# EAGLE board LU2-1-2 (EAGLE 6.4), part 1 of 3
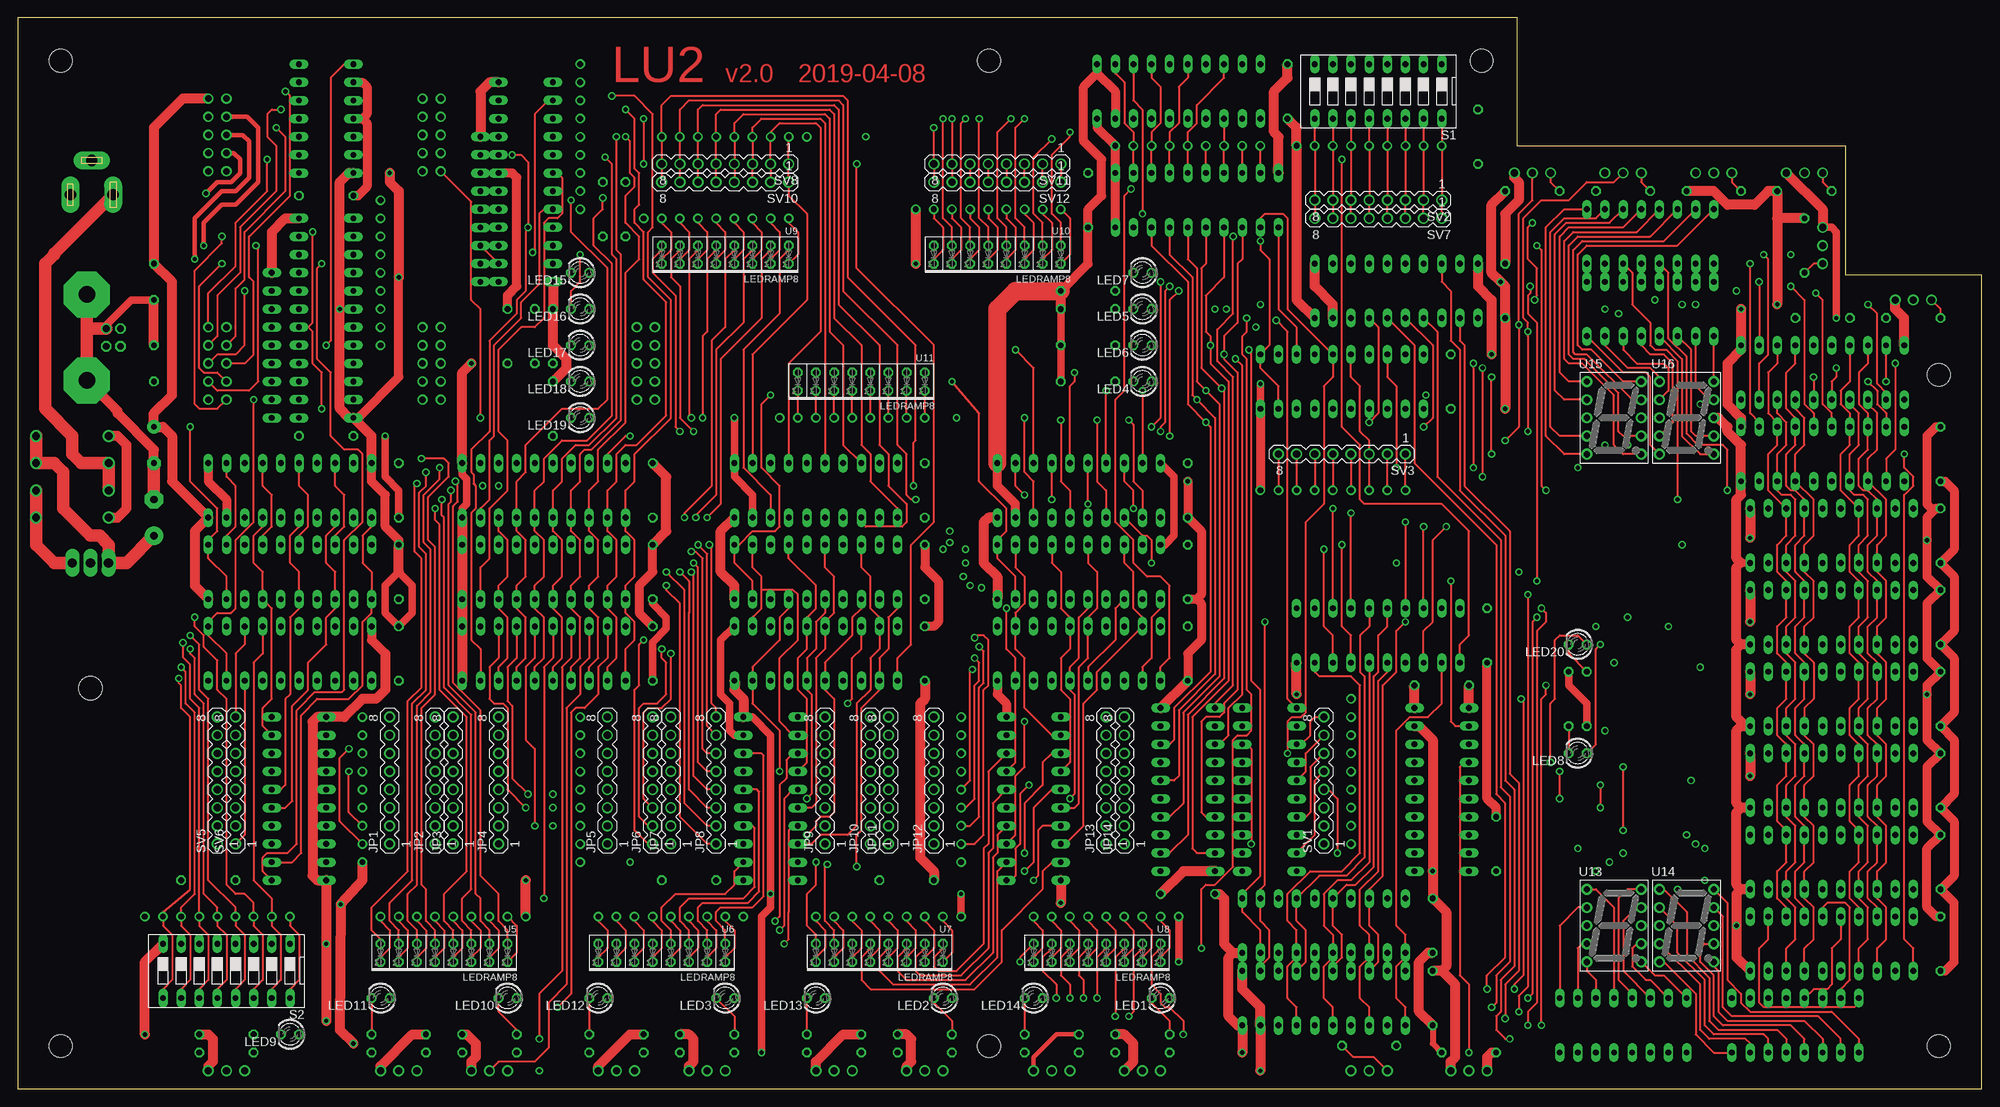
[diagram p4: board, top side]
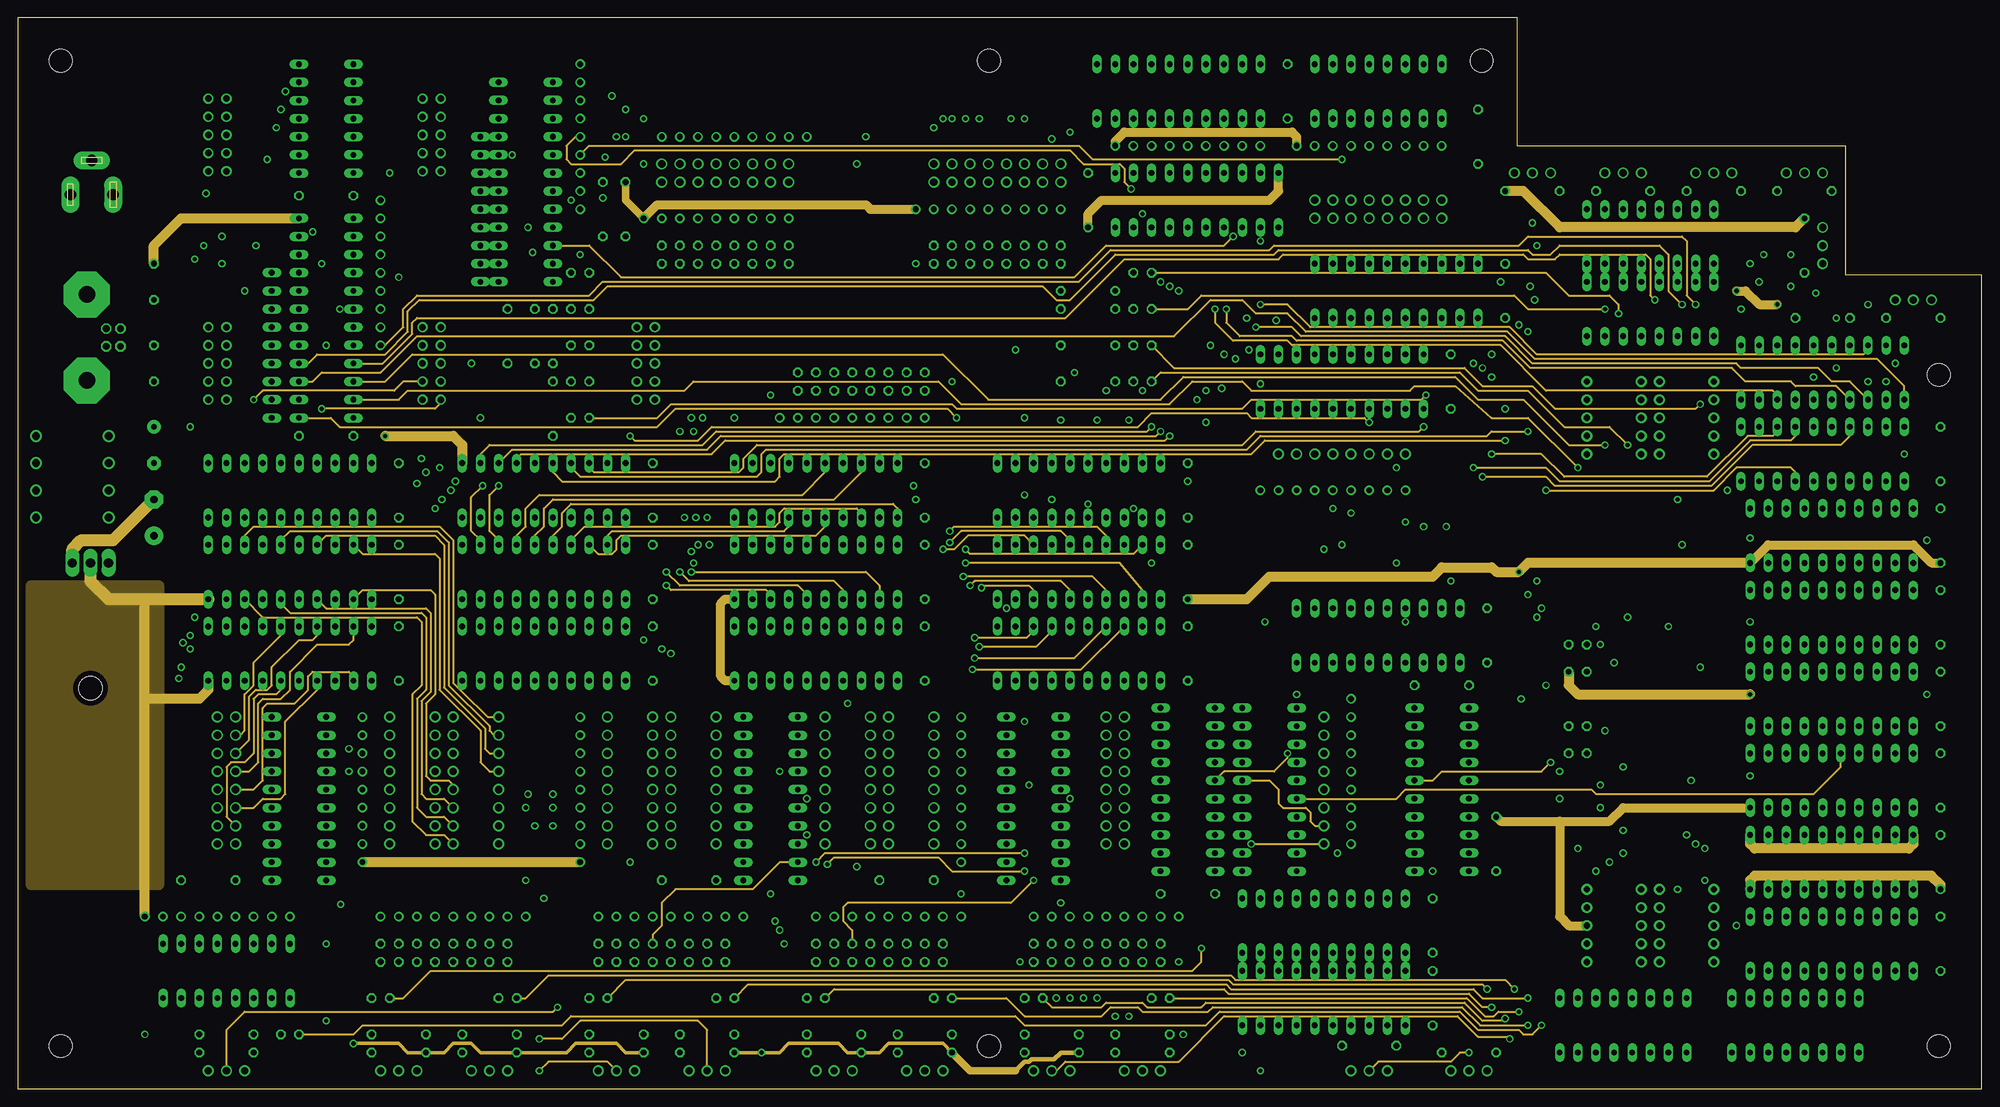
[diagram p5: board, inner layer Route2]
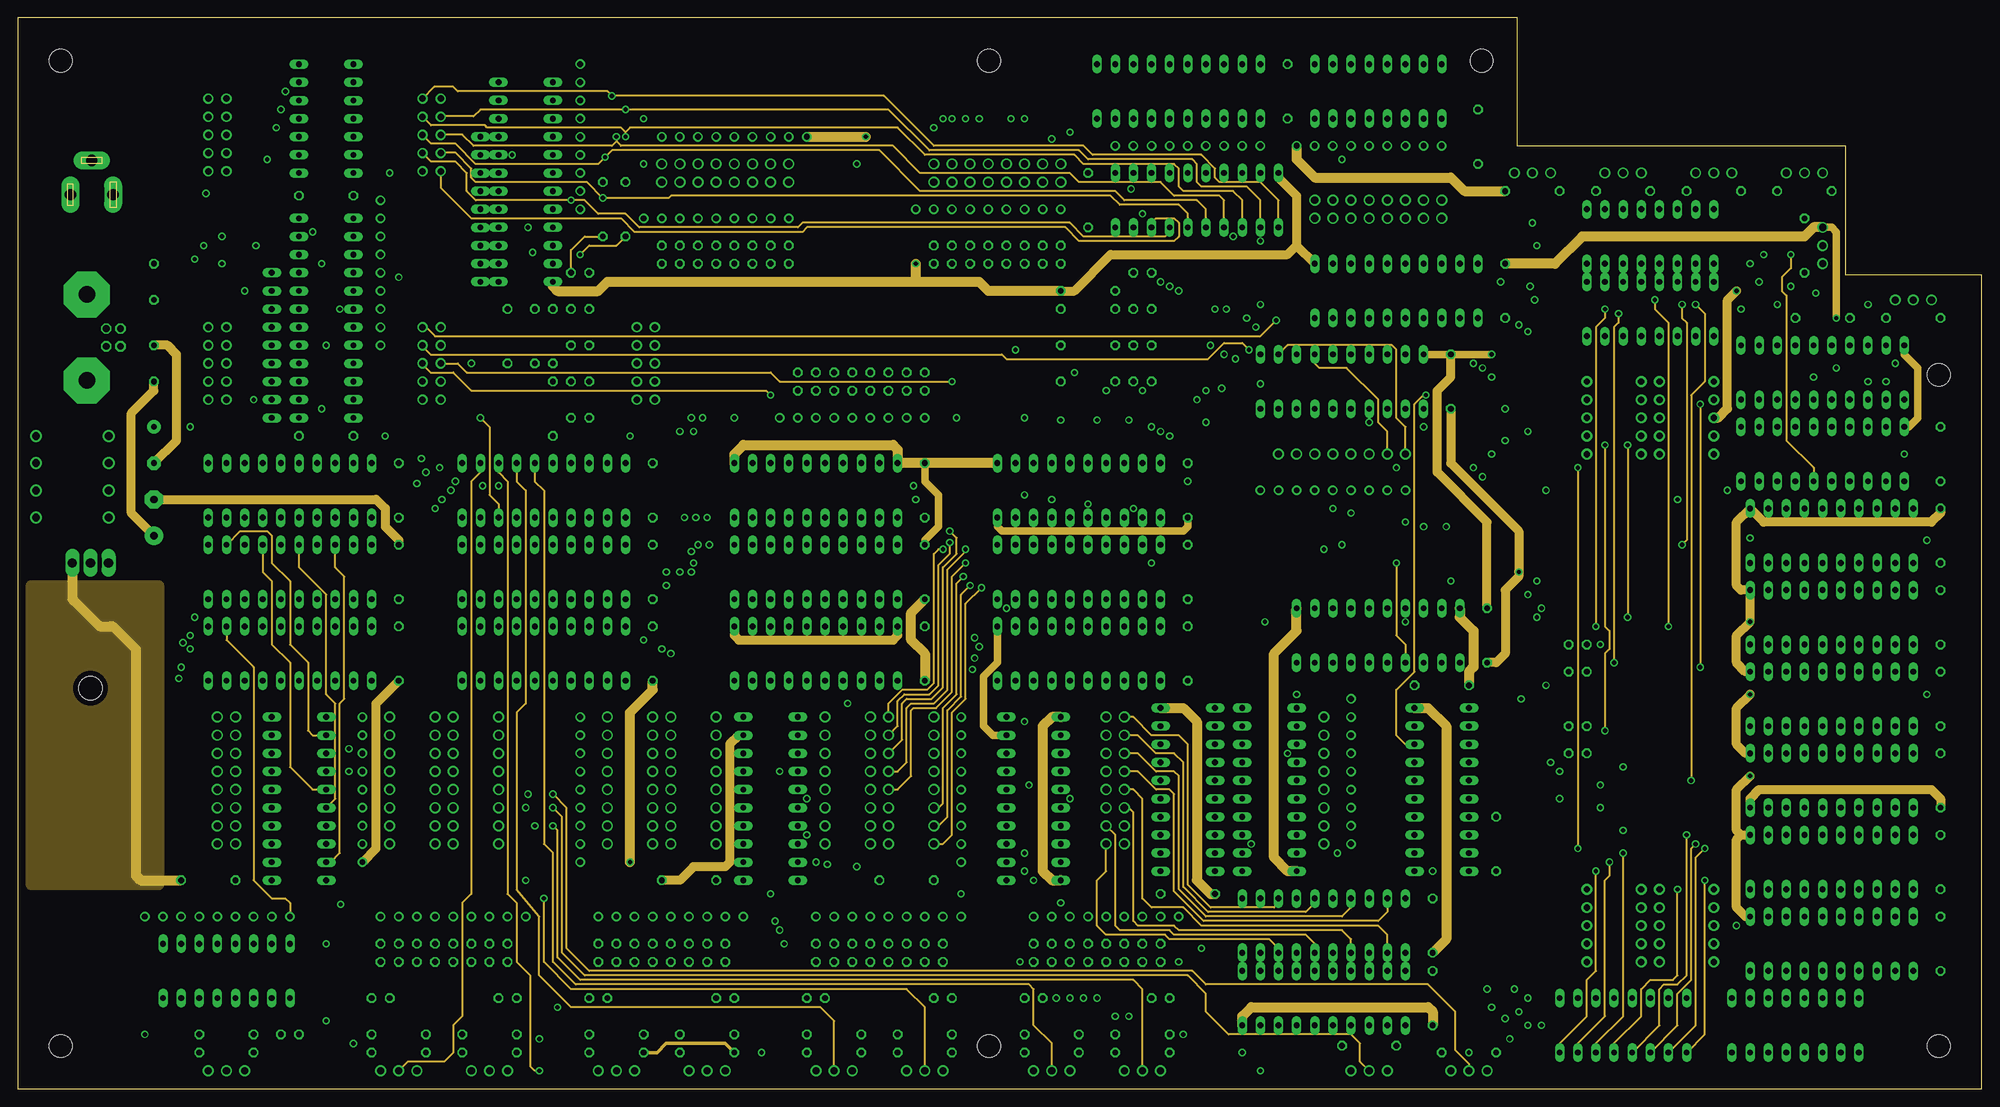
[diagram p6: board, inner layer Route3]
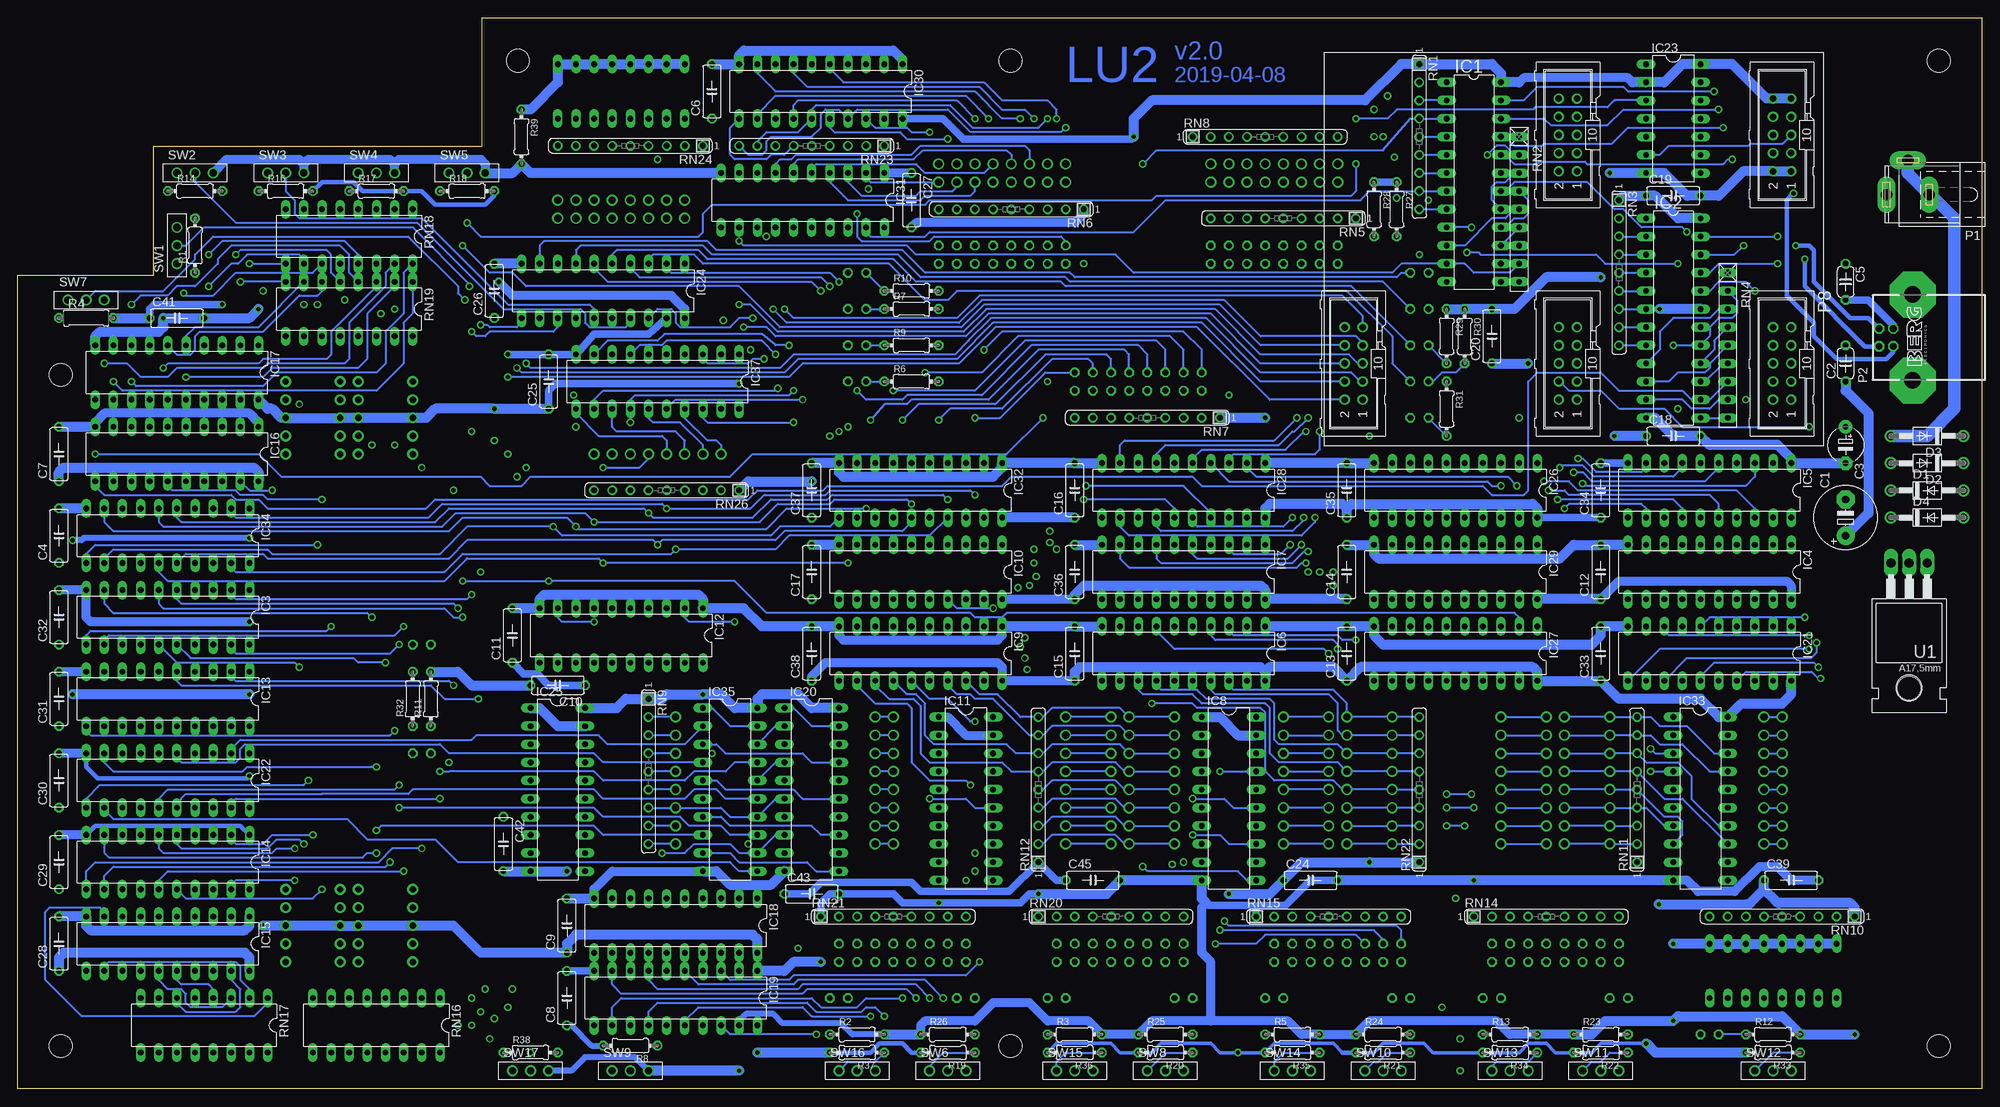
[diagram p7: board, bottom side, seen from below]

Size 275 x 150 mm. Coordinates in mm from the lower left corner, seen from the top.
Outline: 0,0 275,0 275,114 256,114 256,132 210,132 210,150 0,150 0,0
Copper layers (1+2*3+16): Top 0.035mm / dielectric 0.3mm / Route2 0.035mm / dielectric 0.9mm / Route3 0.035mm / dielectric 0.3mm / Bottom 0.035mm
Design rules "default *": minimum track width 10mil, minimum drill 22mil, track to track 10mil, track to pad 10mil, pad to pad 10mil, via to via 10mil, smd to smd 8mil, copper to edge 30mil, drill to drill 8mil, minimum pad ring 10mil, minimum via ring 8mil, stop-mask expansion 4mil, vias tented up to drill 0mil, thermal gap 10mil
Holes 3.2 mm at 6,6 6,144 205,144 269,6 136,6 136,144 269,100
tKeepout: area 0,27.9 to 20.3,71.1

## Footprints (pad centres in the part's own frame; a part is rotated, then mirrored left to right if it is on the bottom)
E5-8,5 = drill 1.016 pad 2.54: + -2.54,0 | drill 1.016 pad 2.54 octagon: - 2.54,0
C050-024X044 = drill 0.813 octagon: 1 -2.54,0; 2 2.54,0
E5-5 = drill 0.813 pad 1.905: + -2.54,0 | drill 0.813 pad 1.905 octagon: - 2.54,0
C313 = drill 0.813 octagon: 1 -3.81,0; 2 3.81,0
DO41-10 = drill 1.118: A 5.08,0; C -5.08,0
DIL24-3 = drill 0.813 long: 1 -13.97,-3.81; 2 -11.43,-3.81; 3 -8.89,-3.81; 4 -6.35,-3.81; 5 -3.81,-3.81; 6 -1.27,-3.81; 7 1.27,-3.81; 8 3.81,-3.81; 9 6.35,-3.81; 10 8.89,-3.81; 11 11.43,-3.81; 12 13.97,-3.81; 13 13.97,3.81; 14 11.43,3.81; 15 8.89,3.81; 16 6.35,3.81; 17 3.81,3.81; 18 1.27,3.81; 19 -1.27,3.81; 20 -3.81,3.81; 21 -6.35,3.81; 22 -8.89,3.81; 23 -11.43,3.81; 24 -13.97,3.81
DIL20 = drill 0.813 long: 1 -11.43,-3.81; 2 -8.89,-3.81; 3 -6.35,-3.81; 4 -3.81,-3.81; 5 -1.27,-3.81; 6 1.27,-3.81; 7 3.81,-3.81; 8 6.35,-3.81; 9 8.89,-3.81; 10 11.43,-3.81; 11 11.43,3.81; 12 8.89,3.81; 13 6.35,3.81; 14 3.81,3.81; 15 1.27,3.81; 16 -1.27,3.81; 17 -3.81,3.81; 18 -6.35,3.81; 19 -8.89,3.81; 20 -11.43,3.81
DIL14 = drill 0.813 long: 1 -7.62,-3.81; 2 -5.08,-3.81; 3 -2.54,-3.81; 4 0,-3.81; 5 2.54,-3.81; 6 5.08,-3.81; 7 7.62,-3.81; 8 7.62,3.81; 9 5.08,3.81; 10 2.54,3.81; 11 0,3.81; 12 -2.54,3.81; 13 -5.08,3.81; 14 -7.62,3.81
MA08R-1 = drill 1.016: 1 -8.89,0; 2 -6.35,0; 3 -3.81,0; 4 -1.27,0; 5 1.27,0; 6 3.81,0; 7 6.35,0; 8 8.89,0
LED3MM = drill 0.813 octagon: A -1.27,0; K 1.27,0
DC21CLIFF = drill 1.6 pad 2.54 long: 1 0.81,0; 2 3.81,-4.8; 3 6.81,0
1729-S = drill 0.95 octagon: 1 1.25,5.98; 2 -1.25,5.98; 3 -1.25,3.98; 4 1.25,3.98 | drill 2.3 pad 6.452 octagon: S1 -6.02,1.27; S2 6.02,1.27
ARM_CTRL = drill 0.914: 1 5.08,1.27; 2 5.08,-1.27; 3 2.54,1.27; 4 2.54,-1.27; 5 0,1.27; 6 0,-1.27; 7 -2.54,1.27; 8 -2.54,-1.27; 9 -5.08,1.27; 10 -5.08,-1.27; 11 -26.92,1.27; 12 -26.92,-1.27; 13 -29.46,1.27; 14 -29.46,-1.27; 15 -32,1.27; 16 -32,-1.27; 17 -34.54,1.27; 18 -34.54,-1.27; 19 -37.08,1.27; 20 -37.08,-1.27; 21 -26.92,-28.73; 22 -26.92,-31.27; 23 -29.46,-28.73; 24 -29.46,-31.27; 25 -32,-28.73; 26 -32,-31.27; 27 -34.54,-28.73; 28 -34.54,-31.27; 29 -37.08,-28.73; 30 -37.08,-31.27; 31 5.08,-28.73; 32 5.08,-31.27; 33 2.54,-28.73; 34 2.54,-31.27; 35 0,-28.73; 36 0,-31.27; 37 -2.54,-28.73; 38 -2.54,-31.27; 39 -5.08,-28.73; 40 -5.08,-31.27; 41 5.08,-58.73; 42 5.08,-61.27; 43 2.54,-58.73; 44 2.54,-61.27; 45 0,-58.73; 46 0,-61.27; 47 -2.54,-58.73; 48 -2.54,-61.27; 49 -5.08,-58.73; 50 -5.08,-61.27
0204/7 = drill 0.813 octagon: 1 -3.81,0; 2 3.81,0
0207/7 = drill 0.813 octagon: 1 -3.81,0; 2 3.81,0
SIL9R = drill 0.813: 1 -10.16,0; 2 -7.62,0; 3 -5.08,0; 4 -2.54,0; 5 0,0; 6 2.54,0; 7 5.08,0; 8 7.62,0; 9 10.16,0
RN-9 = drill 0.813 long: 1 -10.16,0; 2 -7.62,0; 3 -5.08,0; 4 -2.54,0; 5 0,0; 6 2.54,0; 7 5.08,0; 8 7.62,0; 9 10.16,0
DIL16 = drill 0.813 long: 1 -8.89,-3.81; 2 -6.35,-3.81; 3 -3.81,-3.81; 4 -1.27,-3.81; 5 1.27,-3.81; 6 3.81,-3.81; 7 6.35,-3.81; 8 8.89,-3.81; 9 8.89,3.81; 10 6.35,3.81; 11 3.81,3.81; 12 1.27,3.81; 13 -1.27,3.81; 14 -3.81,3.81; 15 -6.35,3.81; 16 -8.89,3.81
DS-08 = drill 0.813 long: 1 -8.89,-3.81; 2 -6.35,-3.81; 3 -3.81,-3.81; 4 -1.27,-3.81; 5 1.27,-3.81; 6 3.81,-3.81; 7 6.35,-3.81; 8 8.89,-3.81; 9 8.89,3.81; 10 6.35,3.81; 11 3.81,3.81; 12 1.27,3.81; 13 -1.27,3.81; 14 -3.81,3.81; 15 -6.35,3.81; 16 -8.89,3.81
SWITCH_DV = drill 1: 1 -2.54,0; 2 0,0; 3 2.54,0
TO220AH = drill 1.3 long: D 0,-10.16; G -2.54,-10.16; S 2.54,-10.16 | hole 3.302: 0,7.366
LEDRAMP8 = drill 0.813 octagon: A0 -8.89,-1.27; A1 -6.35,-1.27; A2 -3.81,-1.27; A3 -1.27,-1.27; A4 1.27,-1.27; A5 3.81,-1.27; A6 6.35,-1.27; A7 8.89,-1.27; K0 -8.89,1.27; K1 -6.35,1.27; K2 -3.81,1.27; K3 -1.27,1.27; K4 1.27,1.27; K5 3.81,1.27; K6 6.35,1.27; K7 8.89,1.27
LED7SEG = drill 0.9 pad 1.5: 1 -3.81,5.08; 2 -3.81,2.54; 3 -3.81,0; 4 -3.81,-2.54; 5 -3.81,-5.08; 6 3.81,-5.08; 7 3.81,-2.54; 8 3.81,0; 9 3.81,2.54; 10 3.81,5.08

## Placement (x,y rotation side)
C1  100u/50V  [E5-8,5]  19.05,80.01 90 bottom
C2  100n  [C050-024X044]  19.05,101.6 90 bottom
C3  4,7u 6V  [E5-5]  19.05,90.17 270 bottom
C4  0,1u  [C313]  269.24,77.47 90 bottom
C5  100n  [C050-024X044]  19.05,113.03 270 bottom
C6  0,1u  [C313]  177.8,139.7 90 bottom
C7  100n  [C313]  269.24,88.9 90 bottom
C8  100n  [C313]  198.12,12.7 90 bottom
C9  0,1u  [C313]  198.12,22.86 90 bottom
C10  0,1u  [C313]  199.39,56.52 180 bottom
C11  0,1u  [C313]  205.74,63.5 90 bottom
C12  0,1u  [C313]  53.34,72.39 90 bottom
C13  0,1u  [C313]  88.9,60.96 90 bottom
C14  0,1u  [C313]  88.9,72.39 90 bottom
C15  0,1u  [C313]  127,60.96 90 bottom
C16  0,1u  [C313]  127,83.82 90 bottom
C17  0,1u  [C313]  163.83,72.39 90 bottom
C18  0,1u  [C313]  43.18,91.44 0 bottom
C19  0,1u  [C313]  43.18,125.09 0 bottom
C20  0,1u  [C313]  68.58,105.41 90 bottom
C24  0,1u  [C313]  93.98,29.21 0 bottom
C25  0,1u  [C313]  200.66,99.06 90 bottom
C26  0,1u  [C313]  208.28,111.76 90 bottom
C27  0,1u  [C313]  149.86,124.46 270 bottom
C28  0,1u  [C313]  269.24,20.32 90 bottom
C29  0,1u  [C313]  269.24,31.75 90 bottom
C30  0,1u  [C313]  269.24,43.18 90 bottom
C31  0,1u  [C313]  269.24,54.61 90 bottom
C32  0,1u  [C313]  269.24,66.04 90 bottom
C33  0,1u  [C313]  53.34,60.96 90 bottom
C34  0,1u  [C313]  53.34,83.82 90 bottom
C35  0,1u  [C313]  88.9,83.82 90 bottom
C36  0,1u  [C313]  127,72.39 90 bottom
C37  0,1u  [C313]  163.83,83.82 90 bottom
C38  0,1u  [C313]  163.83,60.96 90 bottom
C39  0,1u  [C313]  26.67,29.21 0 bottom
C41  0,1u  [C313]  252.73,107.95 0 bottom
C42  0,1u  [C313]  207.01,34.29 270 bottom
C43  0,1u  [C313]  163.83,27.3 0 bottom
C45  0,1u  [C313]  124.46,29.21 0 bottom
D1  1N4004  [DO41-10]  7.62,83.82 0 bottom
D2  1N4004  [DO41-10]  7.62,87.63 180 bottom
D3  1N4004  [DO41-10]  7.62,91.44 180 bottom
D4  1N4004  [DO41-10]  7.62,80.01 0 bottom
IC1  74154E  [DIL24-3]  71.12,127 270 bottom
IC2  74154E  [DIL24-3]  43.18,107.95 270 bottom
IC3  74HC374N  [DIL20]  254,66.04 180 bottom
IC4  SN74BCT760  [DIL20]  38.1,72.39 180 bottom
IC5  74AC244N  [DIL20]  38.1,83.82 180 bottom
IC6  74HC374N  [DIL20]  111.76,60.96 180 bottom
IC7  SN74BCT760  [DIL20]  111.76,72.39 180 bottom
IC8  74AC244N  [DIL20]  105.41,40.64 270 bottom
IC9  74HC374N  [DIL20]  148.59,60.96 180 bottom
IC10  SN74BCT760  [DIL20]  148.59,72.39 180 bottom
IC11  74AC244N  [DIL20]  142.24,40.64 270 bottom
IC12  74HC374N  [DIL20]  190.5,63.5 180 bottom
IC13  74HC374N  [DIL20]  254,54.61 180 bottom
IC14  74HC374N  [DIL20]  254,31.75 180 bottom
IC15  74HC374N  [DIL20]  254,20.32 180 bottom
IC16  74HC374N  [DIL20]  252.73,88.9 180 bottom
IC17  74HC374N  [DIL20]  252.73,100.33 180 bottom
IC18  SN74BCT760  [DIL20]  182.88,22.86 180 bottom
IC19  74AC244N  [DIL20]  182.88,12.7 180 bottom
IC20  74HCT244N  [DIL20]  163.83,41.91 270 bottom
IC21  SN74BCT760  [DIL20]  38.1,60.96 180 bottom
IC22  74HC374N  [DIL20]  254,43.18 180 bottom
IC23  74HC74N  [DIL14]  43.18,135.89 270 bottom
IC24  74AC244N  [DIL20]  193.04,111.76 180 bottom
IC25  74AC244N  [DIL20]  199.39,41.91 270 bottom
IC26  74HC245N  [DIL20]  73.66,83.82 180 bottom
IC27  74HC245N  [DIL20]  73.66,60.96 180 bottom
IC28  74HC244N  [DIL20]  111.76,83.82 180 bottom
IC29  74HC245N  [DIL20]  73.66,72.39 180 bottom
IC30  74HC244N  [DIL20]  162.56,139.7 180 bottom
IC31  74HC245N  [DIL20]  165.1,124.46 180 bottom
IC32  74HC244N  [DIL20]  148.59,83.82 180 bottom
IC33  74HC374N  [DIL20]  39.37,40.64 270 bottom
IC34  74HCT374N  [DIL20]  254,77.47 180 bottom
IC35  SN74BCT760  [DIL20]  175.26,41.91 270 bottom
IC37  74HCT244N  [DIL20]  185.42,99.06 180 bottom
JP1  [MA08R-1]  52.07,43.18 90 top
JP2  [MA08R-1]  58.42,43.18 90 top
JP3  [MA08R-1]  60.96,43.18 90 top
JP4  [MA08R-1]  67.31,43.18 90 top
JP5  [MA08R-1]  82.55,43.18 90 top
JP6  [MA08R-1]  88.9,43.18 90 top
JP7  [MA08R-1]  91.44,43.18 90 top
JP8  [MA08R-1]  97.79,43.18 90 top
JP9  [MA08R-1]  113.03,43.18 90 top
JP10  [MA08R-1]  119.38,43.18 90 top
JP11  [MA08R-1]  121.92,43.18 90 top
JP12  [MA08R-1]  128.27,43.18 90 top
JP13  [MA08R-1]  152.4,43.18 90 top
JP14  [MA08R-1]  154.94,43.18 90 top
LED1  RED  [LED3MM]  160.02,12.7 180 top
LED2  RED  [LED3MM]  129.54,12.7 180 top
LED3  RED  [LED3MM]  99.06,12.7 180 top
LED4  RED  [LED3MM]  157.48,99.06 180 top
LED5  RED  [LED3MM]  157.48,109.22 180 top
LED6  RED  [LED3MM]  157.48,104.14 180 top
LED7  RED  [LED3MM]  157.48,114.3 180 top
LED8  RED  [LED3MM]  218.44,46.99 180 top
LED9  RED  [LED3MM]  38.1,7.62 180 top
LED10  RED  [LED3MM]  68.58,12.7 180 top
LED11  LDA  [LED3MM]  50.8,12.7 180 top
LED12  LDB  [LED3MM]  81.28,12.7 180 top
LED13  LDT  [LED3MM]  111.76,12.7 180 top
LED14  LDR  [LED3MM]  142.24,12.7 180 top
LED15  F3  [LED3MM]  78.74,114.3 180 top
LED16  F2  [LED3MM]  78.74,109.22 180 top
LED17  F1  [LED3MM]  78.74,104.14 180 top
LED18  F0  [LED3MM]  78.74,99.06 180 top
LED19  Cin  [LED3MM]  78.74,93.98 180 top
LED20  MW  [LED3MM]  218.44,62.23 180 top
P1  DC21-PCB16  [DC21CLIFF]  6.53,125.24 180 bottom
P2  USB-NORMAL-S  [1729-S]  8.4,105.23 90 bottom
P8  ARM_CONTROL  [ARM_CTRL]  27.94,101.6 270 bottom
R1  10k  [0204/7]  250.19,118.11 90 bottom
R2  [0204/7]  157.48,7.62 0 bottom
R3  [0204/7]  127,7.62 0 bottom
R4  10k  [0207/7]  265.43,107.95 0 bottom
R5  [0204/7]  96.52,7.62 0 bottom
R6  [0204/7]  149.86,99.06 0 bottom
R7  [0204/7]  149.86,109.22 0 bottom
R8  10k  [0204/7]  189.23,6.03 180 bottom
R9  [0204/7]  149.86,104.14 0 bottom
R10  [0204/7]  149.86,111.76 0 bottom
R11  [0204/7]  217.17,54.61 90 bottom
R12  [0204/7]  29.21,7.62 0 bottom
R13  [0204/7]  66.04,7.62 0 bottom
R14  10k  [0204/7]  250.19,125.73 0 bottom
R16  10k  [0204/7]  237.49,125.73 0 bottom
R17  10k  [0204/7]  224.79,125.73 0 bottom
R18  10k  [0204/7]  212.09,125.73 0 bottom
R19  10k  [0204/7]  144.78,5.08 180 bottom
R20  10k  [0204/7]  114.3,5.08 180 bottom
R21  10k  [0204/7]  83.82,5.08 180 bottom
R22  10k  [0204/7]  53.34,5.08 180 bottom
R23  [0204/7]  53.34,7.62 0 bottom
R24  [0204/7]  83.82,7.62 0 bottom
R25  [0204/7]  114.3,7.62 0 bottom
R26  [0204/7]  144.78,7.62 0 bottom
R27  [0204/7]  81.92,123.19 270 bottom
R28  [0204/7]  85.09,123.19 270 bottom
R29  [0204/7]  74.93,105.41 270 bottom
R30  [0204/7]  72.39,105.41 270 bottom
R31  [0204/7]  74.93,95.25 270 bottom
R32  [0204/7]  219.71,54.61 90 bottom
R33  10k  [0204/7]  29.21,5.08 180 bottom
R34  10k  [0204/7]  66.04,5.08 180 bottom
R35  10k  [0204/7]  96.52,5.08 180 bottom
R36  10k  [0204/7]  127,5.08 180 bottom
R37  10k  [0204/7]  157.48,5.08 180 bottom
R38  10k  [0204/7]  203.2,5.08 0 bottom
R39  27  [0204/7]  204.47,133.35 270 bottom
RN1  10k  [SIL9R]  78.74,133.35 270 bottom
RN2  [RN-9]  64.77,123.19 270 bottom
RN3  10k  [SIL9R]  50.8,114.3 270 bottom
RN4  [RN-9]  35.56,104.14 270 bottom
RN5  220R  [SIL9R]  97.79,121.92 180 bottom
RN6  220R  [SIL9R]  135.89,123.19 180 bottom
RN7  220R  [SIL9R]  116.84,93.98 180 bottom
RN8  10k  [SIL9R]  100.33,133.35 0 bottom
RN9  10k  [SIL9R]  186.69,44.45 270 bottom
RN10  10k  [SIL9R]  27.94,24.13 180 bottom
RN11  47k?  [SIL9R]  48.26,41.91 90 bottom
RN12  47k ?  [SIL9R]  132.08,41.91 90 bottom
RN14  220 R  [SIL9R]  60.96,24.13 0 bottom
RN15  220 ?  [SIL9R]  91.44,24.13 0 bottom
RN16  330  [DIL16]  224.79,8.89 180 bottom
RN17  330  [DIL16]  248.92,8.89 180 bottom
RN18  330  [DIL16]  228.6,119.38 180 bottom
RN19  330  [DIL16]  228.6,109.22 180 bottom
RN20  220 ?  [SIL9R]  121.92,24.13 0 bottom
RN21  220 ?  [SIL9R]  152.4,24.13 0 bottom
RN22  47k ?  [SIL9R]  78.74,41.91 90 bottom
RN23  10k  [SIL9R]  163.83,132.08 180 bottom
RN24  10k  [SIL9R]  189.23,132.08 180 bottom
RN26  10k  [SIL9R]  184.15,83.82 180 bottom
S1  [DS-08]  190.5,139.7 180 top
S2  [DS-08]  29.21,16.51 180 top
SV1  [MA08R-1]  182.88,43.18 90 top
SV2  [MA08R-1]  190.5,124.46 180 top
SV3  [MA08R-1]  185.42,88.9 180 top
SV5  [MA08R-1]  27.94,43.18 90 top
SV6  [MA08R-1]  30.48,43.18 90 top
SV7  [MA08R-1]  190.5,121.92 180 top
SV8  MA08R-1  [MA08R-1]  99.06,129.54 180 top
SV10  MA08R-1  [MA08R-1]  99.06,127 180 top
SV11  MA08R-1  [MA08R-1]  137.16,129.54 180 top
SV12  MA08R-1  [MA08R-1]  137.16,127 180 top
SW1  [SWITCH_DV]  252.73,118.11 90 bottom
SW2  [SWITCH_DV]  250.19,128.27 0 bottom
SW3  [SWITCH_DV]  237.49,128.27 0 bottom
SW4  [SWITCH_DV]  224.79,128.27 0 bottom
SW5  [SWITCH_DV]  212.09,128.27 0 bottom
SW6  [SWITCH_DV]  144.78,2.54 0 bottom
SW7  [SWITCH_DV]  265.43,110.49 0 bottom
SW8  [SWITCH_DV]  114.3,2.54 0 bottom
SW9  [SWITCH_DV]  189.23,2.54 0 bottom
SW10  [SWITCH_DV]  83.82,2.54 0 bottom
SW11  [SWITCH_DV]  53.34,2.54 0 bottom
SW12  [SWITCH_DV]  29.21,2.54 0 bottom
SW13  [SWITCH_DV]  66.04,2.54 0 bottom
SW14  [SWITCH_DV]  96.52,2.54 0 bottom
SW15  [SWITCH_DV]  127,2.54 0 bottom
SW16  [SWITCH_DV]  157.48,2.54 0 bottom
SW17  [SWITCH_DV]  203.2,2.54 0 bottom
U1  LM1084-3,3  [TO220AH]  10.16,63.5 180 bottom
U5  LEDRAMP8  [LEDRAMP8]  59.69,19.05 180 top
U6  LEDRAMP8  [LEDRAMP8]  90.17,19.05 180 top
U7  LEDRAMP8  [LEDRAMP8]  120.65,19.05 180 top
U8  LEDRAMP8  [LEDRAMP8]  151.13,19.05 180 top
U9  LEDRAMP8  [LEDRAMP8]  99.06,116.84 180 top
U10  LEDRAMP8  [LEDRAMP8]  137.16,116.84 180 top
U11  LEDRAMP8  [LEDRAMP8]  118.11,99.06 180 top
U13  DATA HIGH  [LED7SEG]  223.52,22.86 0 top
U14  DATA LOW  [LED7SEG]  233.68,22.86 0 top
U15  ADDRESS HIGH  [LED7SEG]  223.52,93.98 0 top
U16  ADDRESS LOW  [LED7SEG]  233.68,93.98 0 top

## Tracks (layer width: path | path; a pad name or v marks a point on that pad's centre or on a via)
ALUR_0  (via drill 0.6)
  Top 0.305: v140.97,83.19 139.7,84.45 IC32.2 | IC12.3 v184.15,81.28
  Bottom 0.305: IC34.2 245.11,80.64 244.47,80.01 217.49,80.01 215.58,81.92 184.78,81.92 v184.15,81.28 172.4,81.28 170.5,83.19 161.93,83.19 161.29,83.82 141.6,83.82 v140.97,83.19
ALUR_1  (via drill 0.6)
  Top 0.305: v144.78,82.55 IC32.4 | IC12.4 v186.69,80.64
  Bottom 0.305: IC34.5 252.73,80.01 252.09,79.38 216.53,79.38 214.63,81.28 187.32,81.28 v186.69,80.64 186.06,80.01 172.09,80.01 169.54,82.55 161.61,82.55 160.97,83.19 145.41,83.19 v144.78,82.55
ALUR_2  (via drill 0.6)
  Top 0.305: v149.86,81.92 IC32.6 | v194.31,79.38 IC12.7
  Bottom 0.305: IC34.6 255.27,79.38 254.63,78.74 215.58,78.74 213.68,80.64 195.58,80.64 v194.31,79.38 171.13,79.38 168.59,81.92 161.29,81.92 160.66,82.55 150.5,82.55 v149.86,81.92
ALUR_3  (via drill 0.6)
  Top 0.305: v156.21,81.28 156.21,83.82 154.94,85.09 IC32.8 | IC12.8 v196.85,78.74
  Bottom 0.305: IC34.9 262.89,79.38 261.62,78.11 214.63,78.11 212.72,80.01 198.12,80.01 v196.85,78.74 196.53,78.42 170.18,78.42 167.32,81.28 v156.21,81.28
ALUR_4  (via drill 0.6)
  Top 0.305: IC12.13 196.85,64.14 198.12,65.41 198.12,76.83 v200.03,78.74
  Bottom 0.305: IC34.12 262.89,74.3 261.62,75.56 240.03,75.56 239.4,74.93 215.9,74.93 212.09,78.74 v200.03,78.74 198.75,77.47 169.54,77.47 168.28,78.74 161.29,78.74 IC32.11
ALUR_5  (via drill 0.6)
  Top 0.305: IC32.13 157.48,77.47 158.12,77.47 158.75,76.83 v158.75,73.66
  Route3 0.305: v193.04,73.66 193.04,63.5 194.31,62.23 IC12.14
  Bottom 0.305: IC34.15 255.27,72.39 254,71.12 215.26,71.12 212.09,74.3 193.68,74.3 v193.04,73.66 v158.75,73.66
ALUR_6  (via drill 0.6)
  Top 0.305: IC12.17 186.69,63.5 185.42,64.77 v185.42,76.2
  Bottom 0.305: IC32.15 149.86,79.38 151.13,78.11 167.64,78.11 168.91,76.83 184.78,76.83 v185.42,76.2 186.06,76.83 212.09,76.83 214.63,74.3 240.03,74.3 240.66,74.93 251.46,74.93 IC34.16
ALUR_7  (via drill 0.6)
  Top 0.305: IC12.18 184.15,63.5 182.88,64.77 v182.88,75.56
  Bottom 0.305: IC32.17 147.32,77.47 167,77.47 168.91,75.56 v182.88,75.56 183.51,74.93 212.72,74.93 215.26,72.39 244.47,72.39 245.11,73.03 IC34.19
CSIN1  (via drill 0.6)
  Top 0.305: IC1.2 74.3,138.43 72.39,136.53 72.39,117.47 v72.07,117.16 | IC33.11 34.29,30.48 34.29,32.38 34.92,33.02 37.78,33.02 39.05,34.29 39.05,51.75 39.05,53.02 39.37,53.34 41.59,55.56 42.86,55.56 45.4,55.56 45.72,55.88 45.72,76.83 48.26,79.38 48.26,88.9 47.62,89.53 45.72,89.53 43.81,91.44 43.81,100.33 41.91,102.23 41.91,114.94 v42.55,115.57
  Bottom 0.305: IC1.2 RN1.3 | v72.07,117.16 70.48,117.16 70.17,116.84 53.98,116.84 52.7,115.57 v42.55,115.57
CSIN2  (via drill 0.6)
  Top 0.305: IC6.11 123.19,60.33 125.09,62.23 125.09,76.2 128.27,79.38 128.27,104.14 117.47,114.94 v117.47,129.54
  Bottom 0.305: IC1.3 RN1.4 80.01,135.89 83.82,131.44 115.57,131.44 v117.47,129.54
CSIN3  (via drill 0.6)
  Top 0.305: IC9.11 160.02,59.05 161.29,60.33 161.29,70.48 160.02,71.75 158.12,71.75 156.21,73.66 156.21,76.83 153.67,79.38 153.67,96.52 154.94,97.79 154.94,125.09 v155.89,126.05
  Route2 0.305: RN1.5 78.11,133.35 76.83,132.08 76.83,130.18 77.47,129.54 84.45,129.54 86.36,131.44 147.32,131.44 149.22,129.54 154.31,129.54 154.94,128.91 154.94,127 v155.89,126.05
  Bottom 0.305: RN1.5 IC1.4
CSIN4  (via drill 0.6)
  Top 0.305: IC12.11 201.93,62.23 203.2,63.5 203.2,78.11 199.39,81.92 188.59,81.92 187.96,82.55 187.96,90.17 185.42,92.71 v185.42,130.18
  Route2 0.305: RN1.6 80.01,132.08 148.59,132.08 150.5,130.18 v185.42,130.18
  Bottom 0.305: RN1.6 IC1.5
CSIN5
  Top 0.305: IC29.19 64.77,73.03 66.04,74.3 66.04,81.28 68.58,83.82 68.58,90.81 67.31,92.08 67.31,103.5 70.48,106.68 72.39,106.68 73.66,107.95 73.66,121.28 74.3,121.92 75.56,121.92 76.2,122.56 76.2,127.64 75.56,128.27 IC1.6
  Bottom 0.305: RN1.7 IC1.6
CSIN6
  Bottom 0.305: IC1.7 RN1.8 85.72,125.73 87,124.46 114.3,124.46 118.75,120.02 147.32,120.02 147.96,119.38 155.57,119.38 156.21,120.02 IC31.19
CSIN7
  Top 0.305: IC1.8 73.66,123.19 73.03,122.56 73.03,112.71 70.48,110.17 70.48,107.95 66.67,104.14 66.67,91.44 66.04,90.81 66.04,82.55 64.77,81.28 IC26.19
  Bottom 0.305: RN1.9 IC1.8
CSIN8  (via drill 0.6)
  Top 0.305: v69.22,130.81 70.48,130.81 71.44,129.79 v71.44,120.65 | 71.44,120.59 v71.44,120.65 | v71.44,120.65 71.12,120.02 71.12,111.76 69.85,110.49 69.85,108.58 66.04,104.78 66.04,92.08 63.5,89.53 63.5,86.36 63.82,86.04 63.82,84.77 64.14,84.45 64.14,81.28 63.5,80.64 63.5,62.87 64.77,61.59 IC27.19
  Bottom 0.305: v69.22,130.81 67.94,132.08 66.67,132.08 65.41,130.81 RN2.2 | v71.44,120.65 IC1.9
CSIN9  (via drill 0.6)
  Top 0.305: IC20.1 167.64,53.98 170.18,56.52 170.18,99.69 167.96,101.92 167.96,106.36 170.18,108.58 v170.18,119.38
  Route2 0.305: IC1.10 80.01,118.11 84.45,113.67 147.96,113.67 152.4,118.11 168.91,118.11 v170.18,119.38
  Bottom 0.305: IC1.10 72.39,118.11 68.58,121.92 66.67,121.92 65.41,123.19 RN2.5 | IC20.1 166.37,53.34 163.83,50.8 IC20.19
CSIN10  (via drill 0.6)
  Top 0.305: IC37.19 176.53,98.42 173.99,100.97 IC37.1 175.26,104.14 175.26,116.2 173.99,117.47 v173.99,118.75
  Bottom 0.305: v173.99,118.75 173.35,118.11 150.5,118.11 149.22,116.84 121.28,116.84 118.75,114.3 82.55,114.3 81.28,115.57 IC1.11 72.39,115.57 71.12,114.3 66.04,114.3 RN2.8
CSIN11
  Bottom 0.305: IC1.13 RN2.9
CSIN12
  Top 0.305: IC1.14 RN2.7
CSIN13
  Bottom 0.305: IC1.15 RN2.6
CSIN14
  Bottom 0.305: IC1.16 66.67,120.65 65.41,121.92 64.14,121.92 63.5,122.56 63.5,124.46 RN2.4
CSIN15
  Bottom 0.305: IC1.17 68.58,124.46 68.58,126.36 67.94,127 66.67,127 65.41,128.27 RN2.3
CSOUT1
  Bottom 0.305: RN3.3 IC2.2
CSOUT2
  Bottom 0.305: RN3.4 IC2.3
CSOUT3
  Bottom 0.305: RN3.5 IC2.4
CSOUT4
  Bottom 0.305: RN3.6 IC2.5
CSOUT5
  Bottom 0.305: RN3.7 IC2.6
CSOUT6
  Bottom 0.305: RN3.8 IC2.7
CSOUT7  (via drill 0.6)
  Route2 0.305: RN3.9 51.44,104.14 53.98,106.68 53.98,109.22 55.88,111.12 80.01,111.12 81.92,113.03 148.59,113.03 153.03,117.47 175.26,117.47 175.9,118.11 210.19,118.11 211.46,119.38 233.04,119.38 233.68,118.75 233.68,111.12 v234.95,109.86
  Route3 0.305: v234.95,109.86 236.22,108.58 236.22,99.06 234.31,97.16 v234.31,43.18
  Bottom 0.305: RN3.9 IC2.8 | IC22.11 265.43,40.64 263.52,42.55 234.95,42.55 v234.31,43.18
CSOUT8  (via drill 0.6)
  Route2 0.305: IC2.9 51.12,101.6 55.24,105.73 55.24,107.31 55.88,107.95 146.69,107.95 154.94,116.2 176.53,116.2 177.16,116.84 210.82,116.84 211.46,116.2 215.26,116.2 215.9,116.84 227.97,116.84 228.6,116.2 228.6,111.12 v229.24,110.49
  Route3 0.305: v229.24,110.49 229.24,109.22 231.14,107.31 v231.14,64.77
  Bottom 0.305: IC2.9 45.09,103.5 45.09,106.05 43.18,107.95 38.1,107.95 36.83,109.22 RN4.3 | IC3.11 265.43,63.5 264.8,64.14 231.78,64.14 v231.14,64.77
CSOUT9  (via drill 0.6)
  Route2 0.305: IC2.10 51.44,99.06 55.24,102.87 129.54,102.87 135.89,96.52 160.02,96.52 163.19,99.69 201.29,99.69 204.47,96.52 210.82,96.52 217.17,90.17 v222.25,90.17
  Route3 0.305: v222.25,90.17 222.25,64.77 222.88,64.14 222.88,61.59 222.25,60.96 v222.25,50.16
  Bottom 0.305: IC2.10 43.81,99.06 42.55,100.33 38.73,100.33 38.1,100.97 38.1,101.6 RN4.5 | IC13.11 265.43,50.16 264.8,49.53 222.88,49.53 v222.25,50.16
CSOUT10  (via drill 0.6)
  Route2 0.305: IC2.11 53.34,96.52 54.61,97.79 93.34,97.79 94.61,99.06 128.91,99.06 132.08,95.89 161.29,95.89 164.47,99.06 171.45,99.06 172.72,97.79 194.94,97.79 195.58,98.42 201.29,98.42 206.38,93.98 211.46,93.98 v218.44,87
  Route3 0.305: v218.44,87 v218.44,33.66
  Bottom 0.305: IC2.11 41.91,96.52 40.64,95.25 38.1,95.25 36.83,96.52 RN4.8 | IC14.11 265.43,30.48 264.16,31.75 224.47,31.75 222.57,33.66 v218.44,33.66
CSOUT11  (via drill 0.6)
  Top 0.305: IC15.11 265.43,19.68 264.16,20.95 264.16,83.19 265.43,84.45 265.43,85.72 264.16,87 v264.16,88.9
  Route2 0.305: IC2.13 43.81,93.98 45.09,92.71 89.53,92.71 92.08,95.25 130.18,95.25 v131.44,93.98
  Bottom 0.305: v264.16,88.9 241.3,88.9 238.12,85.72 210.19,85.72 208.91,84.45 204.47,84.45 203.2,85.72 175.26,85.72 172.09,88.9 136.53,88.9 v131.44,93.98 | IC2.13 RN4.9
CSOUT12
  Bottom 0.305: IC16.11 264.16,84.45 262.89,83.19 245.11,83.19 244.47,82.55 241.3,82.55 240.03,81.28 217.81,81.28 216.53,82.55 172.72,82.55 171.45,83.82 162.24,83.82 161.61,84.45 137.16,84.45 135.89,85.72 110.49,85.72 109.22,84.45 69.85,84.45 68.58,83.19 64.14,83.19 63.5,83.82 63.5,99.06 62.23,100.33 53.34,100.33 50.8,97.79 41.91,97.79 40.64,96.52 IC2.14 38.1,96.52 RN4.7
CSOUT13
  Route2 0.305: IC17.11 264.16,98.42 260.35,102.23 212.41,102.23 208.6,106.05 180.34,106.05 177.8,108.58 173.35,108.58 171.45,110.49 167,110.49 161.93,105.41 55.88,105.41 50.8,100.33 42.55,100.33 41.27,99.06 IC2.15
  Bottom 0.305: IC2.15 38.73,99.06 36.2,101.6 RN4.6
CSOUT14  (via drill 0.6)
  Route2 0.305: IC2.16 40.64,101.6 41.91,102.87 51.44,102.87 54.61,106.05 54.61,108.9 56.2,110.49 80.64,110.49 82.55,112.39 143.51,112.39 145.41,110.49 147.32,110.49 153.67,116.84 175.9,116.84 176.53,117.47 211.46,117.47 212.09,116.84 214.63,116.84 215.9,118.11 229.87,118.11 231.14,116.84 231.14,111.76 v233.04,109.86
  Route3 0.305: v233.04,109.86 233.04,107.95 233.68,107.31 233.68,76.83 v233.04,76.2
  Bottom 0.305: IC2.16 37.47,103.5 37.47,104.78 RN4.4 | IC34.11 265.43,74.93 264.16,76.2 v233.04,76.2
CSOUT15  (via drill 0.6)
  Top 0.305: IC23.1 45.72,143.51 43.81,141.6 43.81,104.78 v43.18,104.14
  Bottom 0.305: v43.18,104.14 IC2.17 38.1,105.41 38.1,106.68 36.83,107.95 34.92,107.95 34.29,108.58 34.29,110.49 RN4.2
GND  (via drill 0.6)
  Top 0.61: R26.1 145.41,7.62 142.24,4.45 SW6.3
  Top 1.016: R11.2 217.17,56.52 219.71,53.98 R32.1 | R7.2 R9.2 R6.2 | IC2.12 46.35,93.98 | IC10.10 160.66,76.2 161.93,77.47 161.93,85.72 IC32.10 | RN21.1 v162.56,17.78 | IC28.19 102.87,83.19 100.33,85.72 IC28.1 v100.33,93.98 | IC6.1 98.42,62.87 98.42,55.24 99.69,53.98 99.69,50.16 100.33,49.53 IC8.19 | RN20.1 v132.08,27.3 | SW1.3 254,120.65 254.63,120.02 v254.63,107.95 | C5.2 15.88,110.49 12.38,107 P2.4 | C33.2 55.24,66.67 55.24,70.48 53.34,72.39 51.44,70.48 51.44,66.67 C33.2
  Top 1.27: IC5.1 26.67,85.09 29.21,82.55 IC5.19 | 9.87,106.48 9.67,106.68 | IC30.1 151.13,142.24 | 151.13,142.24 153.67,139.7 IC30.19 | IC32.19 139.7,81.92 137.16,84.45 IC32.1 | C36.2 127,73.03 128.91,71.12 128.91,65.41 128.27,64.77 C15.2 | C14.2 88.9,72.39 87,70.48 87,66.67 C13.2 | C7.2 268.61,92.71 267.33,91.44 267.33,81.92 267.97,81.28 C4.2 268.61,81.28 267.33,80.01 v267.33,76.83 267.33,71.75 C32.2 267.33,67.94 267.33,60.33 C31.2 267.33,56.52 v267.33,55.24 267.33,48.9 C30.2 267.33,45.09 267.33,37.47 C29.2 267.33,33.66 267.33,25.4 268.61,24.13 C28.2 | R10.2 149.86,115.57 C27.2 149.86,123.19 151.76,125.09 151.76,130.18 149.22,132.72 149.22,140.34 151.13,142.24 | C20.2 68.58,111.12 69.85,112.39 69.85,127.64 69.22,128.27 IC1.19 | C12.2 53.34,76.83 51.44,78.74 51.44,83.19 49.53,85.09 IC5.10 | IC21.10 49.53,62.87 51.44,60.96 | IC2.12 47.62,93.98 53.34,99.69 v53.34,113.67
  Top 1.422: C2.2 C5.2 | C14.2 90.81,78.11 90.81,85.72 C35.2 | 53.34,72.39 C12.2 | C3.- 19.05,89.53 13.97,94.61 13.97,94.93 13.63,95.25 P2.S1 | 199.39,16.51 200.03,17.14 200.03,24.77 C9.2 v198.12,30.48 198.12,48.9 196.22,50.8 IC25.19 | 199.39,16.51 C8.2 | R12.2 26.67,7.62 27.3,6.99 27.3,3.81 26.67,3.17 SW12.3 | SW15.3 124.46,3.17 125.09,3.81 125.09,6.99 124.46,7.62 R3.2 | IC31.10 176.53,133.35 175.9,133.99 175.9,139.7 177.8,141.6 C6.2 | SW5.3 209.55,127.64 210.19,127 210.19,124.46 208.28,122.56 C26.2 | IC25.1 C10.2 | IC17.10 264.16,107.95 262.89,109.22 SW7.3 | IC24.10 204.47,112.39 206.38,110.49 v206.38,102.87 | R7.2 R10.2 | R31.1 76.83,100.97 76.83,102.23 74.93,104.14 R29.1 IC1.12 | IC19.1 171.45,13.97 173.99,11.43 IC19.19 v173.99,2.54 | SW16.3 156.21,3.81 156.21,6.35 154.94,7.62 R2.2 | SW8.3 111.76,3.81 115.57,7.62 R25.1 | SW14.3 93.98,3.17 94.61,3.81 94.61,6.99 93.98,7.62 R5.2 | SW10.3 81.28,3.17 85.72,7.62 R24.1 | R13.2 62.87,7.62 64.14,6.35 64.14,4.45 63.5,3.81 SW13.3 | v17.78,7.62 17.78,17.78 S2.8 | SW11.3 50.8,3.17 55.24,7.62 R23.1 | IC5.10 49.53,91.44 IC2.12 | 46.35,93.98 45.09,95.25 v45.09,109.22 45.09,127 46.35,128.27 IC23.7 | SW17.3 200.66,3.81 201.29,4.45 201.29,14.61 199.39,16.51 | IC20.10 163.19,30.48 C43.2 | v43.18,9.53 v43.18,20.32 IC33.10 41.91,29.21 41.27,29.84 41.27,51.44 41.91,52.07 IC33.1 45.72,52.07 48.26,54.61 50.16,54.61 51.44,55.88 51.44,60.96 | SW2.3 252.73,123.19 SW1.3 | v241.3,109.22 IC17.1 241.3,103.5 239.4,101.6 239.4,95.89 241.3,93.98 IC16.1 | RN14.1 v71.12,29.21 | IC24.19 184.15,109.86 181.61,112.39 IC24.1 | IC22.1 v242.57,43.81 | IC13.1 v242.57,55.24 | IC3.1 v242.57,65.41
  Top 1.422: IC34.1 v242.57,77.15 | v52.07,128.27 52.07,127 53.34,125.73 v53.34,113.67 | IC11.10 v146.05,26.04 | RN6.1 v125.73,115.57
  Top 1.778: C3.- C1.- | D1.A D4.A 2.54,76.2 5.08,73.66 U1.G | P2.S2 9.67,106.68 P2.S1 | P2.4 9.87,106.48
  Top 2.54: IC32.1 137.16,109.22 139.7,111.76 R10.2
  Route2 1.016: R28.1 85.09,124.46 RN5.1
  Route2 1.27: C27.2 149.86,122.56 151.76,124.46 175.26,124.46 176.53,125.73 IC31.10 | RN5.1 89.53,123.83 118.75,123.83 119.38,123.19 RN6.1
  Route2 1.422: R11.2 217.17,56.52 218.44,55.24 v242.57,55.24 | IC14.10 265.43,34.29 264.8,33.66 243.21,33.66 242.57,34.29 IC14.1
  Route2 1.676: U1.G 7.62,75.56 8.89,76.83 13.34,76.83 C1.-
  Route3 1.016: IC17.10 264.16,102.87 266.06,100.97 266.06,93.98 264.8,92.71 IC16.10 | C16.2 127,85.09 128.91,83.19 128.91,78.74 127,76.83 C36.2 | IC9.1 137.16,59.69 135.25,57.78 135.25,50.8 136.53,49.53 IC11.19 | SW1.3 254,120.65 254.63,120.02 v254.63,107.95 | v206.38,102.87 C25.2 IC37.10
  Route3 1.27: IC31.10 176.53,127.64 179.07,125.09 179.07,118.11 | 179.07,118.11 IC24.1 | C11.2 205.74,79.38 198.75,86.36 198.75,97.79 200.66,99.69 C25.2 | IC8.19 100.97,49.53 99.69,48.26 99.69,31.75 99.06,31.11 94.61,31.11 92.71,29.21 C24.2 | IC15.1 241.94,24.13 240.66,25.4 240.66,34.92 241.3,35.56 | 241.3,35.56 IC14.1 | 241.3,35.56 240.66,36.2 240.66,41.91 v242.57,43.81 | IC22.1 241.94,46.99 240.66,48.26 240.66,53.34 v242.57,55.24 | IC13.1 241.94,58.42 240.66,59.69 240.66,63.5 v242.57,65.41 IC3.1 241.3,69.85 240.66,70.48 240.66,79.38 IC34.1 244.47,79.38 267.97,79.38 269.24,80.64 C4.2 | IC6.1 100.33,63.5 100.97,62.87 122.56,62.87 123.19,63.5 IC6.10 | C3.- 22.23,90.81 22.23,102.87 20.95,104.14 C2.2 | R10.2 147.96,111.76 153.03,116.84 177.8,116.84 179.07,118.11 | C1.- 50.16,82.55 51.44,81.28 51.44,78.74 53.34,76.83 C12.2
  Route3 1.422: IC12.10 201.93,66.04 203.84,64.14 203.84,59.05 203.2,58.42 C10.2 | IC28.1 100.33,88.9 101.6,90.17 122.56,90.17 123.19,89.53 IC28.10 IC32.1 | IC11.1 144.78,52.07 143.51,50.8 143.51,30.48 144.78,29.21 IC11.10 | IC35.10 177.8,30.48 175.9,32.38 175.9,60.96 179.07,64.14 IC12.1 | SW1.3 251.46,120.65 250.19,119.38 219.07,119.38 215.26,115.57 C26.2 | IC1.12 74.93,112.39 75.56,111.76 81.28,111.76 82.55,113.03 125.73,113.03 | 125.73,113.03 134.62,113.03 135.89,111.76 R10.2 | U1.G 7.62,68.84 arc45 7.81,68.39 11.43,64.77 13.07,64.77 arc-45 13.52,64.58 16.51,61.59 16.51,30.11 arc45 16.7,29.66 17.14,29.21 C39.2 | v125.73,115.57 125.73,113.03
  Bottom 0.61: IC14.10 264.16,36.83 243.84,36.83 IC14.1 | IC22.10 265.43,45.09 263.84,43.5 242.89,43.5 v242.57,43.81
  Bottom 0.813: SW9.3 188.59,4.45 195.58,4.45 197.49,2.54 SW17.3 | R2.2 158.12,7.62 159.7,9.21 167.96,9.21 169.23,10.48 173.04,10.48 173.99,9.53 IC19.19 | v242.57,77.15 265.75,77.15 266.06,76.83 v267.33,76.83
  Bottom 1.016: IC5.10 C34.2 | v132.08,27.3 133.35,27.3 134.62,26.04 v146.05,26.04 151.13,26.04 152.4,27.3 C43.2 161.29,27.3 162.56,26.04 RN21.1 | v206.38,102.87 C25.2 IC37.10 194.31,105.73 186.69,105.73 IC24.19 | R27.1 R28.1 | P2.4 12.38,107 15.88,110.49 C5.2 | C24.2 93.98,29.21 97.47,25.72 101.28,25.72 101.6,25.4 | RN15.1 101.6,25.4 | 101.6,25.4 101.92,25.72 108.27,25.72 108.58,26.04 | IC19.10 C8.2
  Bottom 1.27: R23.1 R13.2 66.04,7.62 67.94,9.53 85.72,9.53 R24.1 R5.2 95.25,7.62 97.16,9.53 107.95,9.53 | C32.2 IC3.10 265.43,66.04 264.8,65.41 v242.57,65.41 | IC13.10 C31.2 | IC22.10 C30.2 | IC14.10 C29.2 | IC9.10 160.02,63.5 159.38,62.87 137.79,62.87 137.16,63.5 IC9.1 | 151.13,144.15 IC30.1 | SW2.3 245.75,130.18 235.59,130.18 234.95,129.54 | 222.25,129.54 222.88,130.18 234.31,130.18 234.95,129.54 | SW4.3 222.25,129.54 | 222.25,129.54 221.62,130.18 210.19,130.18 209.55,129.54 SW5.3 | IC16.1 241.3,93.34 242.57,94.61 262.89,94.61 264.16,93.34 IC16.10 | C39.2 26.67,29.21 28.57,31.11 31.11,31.11 34.61,27.62 39.69,27.62 41.27,29.21 IC33.10 45.09,29.21 | 107.95,9.53 116.2,9.53 R25.1 R3.2 125.09,9.53 130.81,9.53 133.35,12.06 138.43,12.06 140.97,9.53 147.96,9.53 148.59,8.89 R26.1 | RN6.1 125.73,122.56 127,121.28 149.22,121.28 C27.2 | IC11.1 144.78,52.07 142.24,49.53 IC11.19 | 107.95,9.53 107.95,17.78 109.22,19.05 109.22,25.4 108.58,26.04 | IC18.10 194.31,27.94 191.77,30.48 IC35.10 | 234.95,129.54 SW3.3
  Bottom 1.422: C3.- IC5.1 26.67,88.27 28.57,90.17 38.1,90.17 C18.2 43.18,91.44 45.72,93.98 IC2.12 | P8.11 P8.12 33.41,128.52 36.83,125.09 C19.2 41.27,125.09 44.45,128.27 IC23.7 v52.07,128.27 | S2.8 S2.7 S2.6 S2.5 S2.4 S2.3 S2.2 S2.1 v43.18,20.32 | IC6.1 C13.2 IC27.10 85.09,63.5 83.82,62.23 54.61,62.23 53.34,63.5 C33.2 IC21.10 | IC6.10 C15.2 IC9.1 | C36.2 IC7.10 | IC28.10 C16.2 IC32.1 137.16,87 138.43,85.72 159.38,85.72 160.02,86.36 IC32.10 C37.2 | IC26.10 C35.2 IC28.1 | IC4.10 C12.2 57.15,76.2 59.05,74.3 84.45,74.3 85.09,74.93 IC29.10 C14.2 | v132.08,27.3 122.56,27.3 C45.2 IC8.10 109.22,26.67 108.58,26.04 | IC35.10 177.16,30.48 175.26,28.57 169.54,28.57 IC20.10 | C42.2 IC25.10 v198.12,30.48 | C9.2 IC18.10 | R2.2 R26.1 | IC16.10 C7.2 | IC34.10 C4.2 | C28.2 IC15.10 265.43,22.86 264.8,22.23 243.21,22.23 242.57,22.86 IC15.1 | IC9.10 C38.2 170.81,64.77 173.35,67.31 IC12.1 179.07,68.58 179.71,69.22 201.29,69.22 201.93,68.58 IC12.10 C11.2 | IC10.10 C17.2 | C6.2 IC30.10 173.99,144.78 173.35,145.41 152.4,145.41 151.13,144.15 | SW5.3 205.74,128.27 R39.2 203.2,128.27 IC31.10 | IC25.1 201.93,53.34 199.39,50.8 IC25.19 | R11.2 213.36,58.42 211.46,56.52 C10.2 | IC24.10 C26.2 | R29.1 R30.1 C20.2 65.41,109.22 60.96,113.67 v53.34,113.67 | v173.99,2.54 SW9.3 | v17.78,7.62 R12.2 27.94,10.16 42.55,10.16 v43.18,9.53 52.7,9.53 54.61,7.62 R23.1 | IC2.19 v45.09,109.22 | IC33.10 v71.12,29.21 C24.2 | v162.56,17.78 166.37,17.78 167.64,16.51 IC19.1 | v241.3,109.22 242.57,107.95 C41.2 v254.63,107.95 254.63,106.68 255.27,106.05 263.52,106.05 264.16,105.41 IC17.10 | IC8.1 106.68,52.07 104.14,49.53 IC8.19 | v242.57,55.24 v267.33,55.24
  Bottom 1.422: v100.33,93.98 RN7.1
  pour Route3: 20.32,70.48 20.32,28.57 arc-90 19.68,27.94 1.91,27.94 arc-90 1.27,28.57 1.27,70.48 arc-90 1.91,71.12 19.68,71.12 arc-90
INBUS0  (via drill 0.6)
  Top 0.305: IC27.18 67.31,59.05 68.58,60.33 68.58,66.04 67.31,67.31 IC29.18 67.31,70.48 68.58,71.75 68.58,76.83 67.31,78.11 IC26.18 | IC31.18 158.75,118.11 163.83,113.03 163.83,95.89 v166.37,93.34 167,92.71 167,58.42 161.93,53.34 161.93,48.9 161.29,48.26 IC20.18 | v64.77,93.98 64.77,109.22 63.5,110.49 63.5,124.23 P8.22
  Route3 0.305: IC26.18 67.31,81.92 66.04,83.19 66.04,92.71 v64.77,93.98 | IC31.18 158.75,121.28 159.38,121.92 161.93,121.92 162.56,121.28 162.56,119.38 161.93,118.75 148.59,118.75 146.69,120.65 110.49,120.65 109.86,120.02 86.36,120.02 84.45,121.92 63.5,121.92 59.21,126.21 P8.22
  Bottom 0.305: IC37.18 179.07,93.98 178.44,93.34 v166.37,93.34
INBUS1  (via drill 0.6)
  Top 0.305: IC27.17 69.85,59.05 71.12,60.33 71.12,66.04 69.85,67.31 IC29.17 69.85,70.48 71.12,71.75 71.12,76.83 69.85,78.11 IC26.17 69.85,85.09 71.12,86.36 71.12,90.17 76.2,95.25 81.28,95.25 82.55,96.52 82.55,114.94 77.47,120.02 v77.47,124.46 | IC31.17 161.29,116.84 164.47,113.67 164.47,97.16 v165.1,96.52 167.64,93.98 167.64,58.1 162.56,53.02 162.56,43.81 161.93,43.18 IC20.16
  Route3 0.305: IC31.17 161.29,120.02 160.66,119.38 149.22,119.38 147.32,121.28 109.86,121.28 109.22,120.65 87,120.65 85.09,122.56 81.28,122.56 79.38,124.46 v77.47,124.46 64.14,124.46 62.87,125.73 62.87,128.27 61.28,129.86 57.87,129.86 P8.23
  Bottom 0.305: IC37.16 182.88,96.52 v165.1,96.52
INBUS2  (via drill 0.6)
  Top 0.305: IC27.16 72.39,59.05 73.66,60.33 73.66,66.04 72.39,67.31 IC29.16 72.39,70.48 73.66,71.75 73.66,76.83 72.39,78.11 IC26.16 72.39,83.82 73.66,85.09 73.66,88.27 76.2,90.81 79.69,90.81 83.19,94.3 83.19,115.57 80.64,118.11 80.64,121.92 81.92,123.19 v81.92,124.78 | IC31.16 163.83,116.2 165.1,114.94 165.1,99.06 v166.37,97.79 168.28,95.89 168.28,57.78 163.19,52.7 163.19,40.01 161.29,38.1 IC20.14
  Route3 0.305: IC31.16 163.83,122.56 162.56,123.83 154.31,123.83 153.03,125.09 91.44,125.09 91.12,124.78 v81.92,124.78 79.69,127 64.14,127 63.5,127.64 63.5,128.91 61.28,131.13 59.28,131.13 P8.24
  Bottom 0.305: IC37.14 189.23,96.52 188.59,97.16 167,97.16 v166.37,97.79
INBUS3  (via drill 0.6)
  Top 0.305: IC27.15 74.93,59.05 76.2,60.33 76.2,66.04 74.93,67.31 IC29.15 74.93,70.48 76.2,71.75 76.2,76.83 74.93,78.11 IC26.15 74.93,83.82 76.2,85.09 76.2,88.27 78.11,90.17 80.01,90.17 83.82,93.98 83.82,116.2 83.19,116.84 83.19,129.54 v82.23,130.49 | IC31.15 166.37,115.57 165.74,114.94 165.74,100.97 v168.59,98.11 168.91,97.79 168.91,57.47 163.83,52.39 163.83,35.56 161.29,33.02 IC20.12
  Route3 0.305: IC31.15 166.37,123.19 165.1,124.46 154.94,124.46 153.67,125.73 126.36,125.73 120.65,131.44 83.19,131.44 v82.23,130.49 81.28,129.54 64.14,129.54 61.28,132.4 57.87,132.4 P8.25
  Bottom 0.305: IC37.12 194.31,96.52 193.04,97.79 168.91,97.79 v168.59,98.11
INBUS4  (via drill 0.6)
  Top 0.305: IC27.14 77.47,59.05 78.74,60.33 78.74,66.04 77.47,67.31 IC29.14 77.47,70.48 78.74,71.75 78.74,76.83 77.47,78.11 IC26.14 77.47,83.82 78.74,85.09 78.74,88.9 79.38,89.53 80.33,89.53 84.45,93.66 84.45,116.84 83.82,117.47 v83.82,133.35 | IC31.14 168.91,113.67 166.37,111.12 166.37,106.05 167,105.41 v167,104.14 167,101.6 169.54,99.06 169.54,57.15 164.47,52.07 164.47,33.66 165.1,33.02 IC20.9
  Route3 0.305: IC31.14 168.91,124.46 168.28,125.09 161.93,125.09 160.02,127 148.59,127 147.32,128.27 126.36,128.27 122.56,132.08 84.45,132.08 83.82,132.72 | 83.82,132.72 83.19,132.08 63.82,132.08 62.23,133.67 59.28,133.67 P8.26 | v83.82,133.35 83.82,132.72
  Bottom 0.305: v167,104.14 168.91,104.14 170.81,105.73 184.47,105.73 185.42,104.78 192.41,104.78 IC37.9
INBUS5  (via drill 0.6)
  Top 0.305: IC27.13 80.01,59.05 81.28,60.33 81.28,66.04 80.01,67.31 IC29.13 80.01,70.48 81.28,71.75 81.28,76.83 80.01,78.11 IC26.13 80.01,83.82 81.28,85.09 81.28,89.53 85.09,93.34 85.09,114.3 87,116.2 87,119.38 85.09,121.28 85.09,125.09 86.36,126.36 86.36,127.64 85.72,128.27 85.72,132.72 v85.09,133.35 | IC31.13 171.45,116.2 170.81,115.57 170.81,107.31 168.91,105.41 v168.91,102.87 168.91,102.23 170.81,100.33 170.81,55.88 168.91,53.98 168.91,52.7 168.28,52.07 166.37,52.07 165.74,51.44 165.74,38.73 166.37,38.1 IC20.7
  Route3 0.305: IC31.13 171.45,124.46 170.18,125.73 163.19,125.73 162.56,126.36 162.56,128.91 161.93,129.54 149.22,129.54 147.96,130.81 127,130.81 123.19,134.62 85.72,134.62 85.09,133.99 | 85.09,133.99 84.45,134.62 65.72,134.62 65.41,134.94 57.87,134.94 P8.27 | v85.09,133.35 85.09,133.99
  Bottom 0.305: v168.91,102.87 170.81,104.78 184.15,104.78 184.78,104.14 187.96,104.14 IC37.7
INBUS6  (via drill 0.6)
  Top 0.305: IC27.12 82.55,59.05 83.82,60.33 83.82,66.04 82.55,67.31 IC29.12 82.55,70.48 83.82,71.75 83.82,76.83 82.55,78.11 IC26.12 82.55,83.82 83.82,85.09 83.82,88.9 85.09,90.17 86.68,90.17 90.81,94.3 90.81,110.17 87.63,113.35 87.63,120.02 86.36,121.28 86.36,123.19 87,123.83 87,128.27 86.36,128.91 86.36,135.89 v85.09,137.16 | IC31.12 173.99,121.92 174.62,122.56 177.16,122.56 177.8,121.92 177.8,109.22 IC37.5 184.15,99.69 182.88,98.42 182.88,81.92 180.34,79.38 180.34,52.7 179.71,52.07 178.44,52.07 177.8,51.44 v177.8,46.99
  Route2 0.305: v177.8,46.99 177.8,46.35 175.9,44.45 168.91,44.45 IC20.5
  Route3 0.305: IC31.12 173.99,124.46 172.09,126.36 165.74,126.36 165.1,127 165.1,129.54 164.47,130.18 149.86,130.18 148.59,131.44 127.64,131.44 121.92,137.16 v85.09,137.16 64.77,137.16 63.82,136.21 59.28,136.21 P8.28
INBUS7  (via drill 0.6)
  Top 0.305: IC27.11 85.09,61.59 86.36,62.87 86.36,65.41 85.09,66.67 IC29.11 85.09,70.48 86.36,71.75 86.36,76.83 85.09,78.11 IC26.11 85.09,83.82 86.36,85.09 86.36,88.9 91.44,93.98 91.44,110.49 88.27,113.67 88.27,120.02 88.9,120.65 88.9,136.53 86.36,139.06 v83.19,139.06 | IC31.11 176.53,109.22 179.07,106.68 IC37.3 | IC20.3 168.28,48.26 169.54,49.53 169.54,53.34 171.45,55.24 171.45,101.28 v170.5,102.23
  Route3 0.305: IC31.11 176.53,124.46 173.99,127 168.28,127 167.64,127.64 167.64,128.91 165.74,130.81 150.5,130.81 149.22,132.08 128.27,132.08 121.28,139.06 v83.19,139.06 82.55,139.7 61.59,139.7 60.96,140.34 58.33,140.34 P8.29
  Bottom 0.305: v170.5,102.23 172.09,102.23 172.72,101.6 178.44,101.6 179.07,102.23 IC37.3
IRQ
  Bottom 0.305: IC23.6 45.09,130.81 43.81,132.08 32.7,132.08 32.38,132.4 27.87,132.4 P8.15
N$1  (via drill 0.6)
  Top 0.305: v213.36,8.89 213.36,54.61 214,55.24 v214,56.52
  Route2 0.305: LED9.A 46.99,7.62 48.26,8.89 76.2,8.89 77.47,10.16 139.7,10.16 140.97,8.89 166.37,8.89 168.28,10.79 201.93,10.79 204.47,8.26 210.19,8.26 210.82,7.62 212.09,7.62 v213.36,8.89
  Bottom 0.305: IC13.2 245.11,57.78 244.47,57.15 214.63,57.15 v214,56.52
N$2  (via drill 0.6)
  Top 0.305: IC27.9 82.55,60.33 81.28,59.05 81.28,55.24 79.38,53.34 78.11,53.34 77.47,52.7 77.47,13.34 v75.56,11.43
  Route2 0.305: SW12.2 29.21,8.26 31.75,10.79 74.93,10.79 v75.56,11.43
N$3  (via drill 0.6)
  Top 0.305: v210.5,54.61 210.82,54.29 210.82,15.88 209.55,14.61 v209.55,13.97
  Route2 0.305: LED10.A 71.12,12.7 74.3,15.88 169.86,15.88 170.5,15.24 208.28,15.24 v209.55,13.97
  Bottom 0.305: IC13.5 252.73,57.15 252.09,56.52 217.17,56.52 215.26,54.61 v210.5,54.61
N$4  (via drill 0.6)
  Top 0.305: LED8.A 220.98,48.26 220.98,61.59 v221.62,62.23
  Bottom 0.305: IC3.19 245.11,61.59 244.47,60.96 222.88,60.96 v221.62,62.23
N$5  (via drill 0.6)
  Route2 0.305: LED7.A 214,114.3 217.17,111.12 222.88,111.12 224.16,109.86 v224.16,108.58
  Route3 0.305: v224.16,108.58 224.16,107.31 223.52,106.68 v223.52,59.69
  Bottom 0.305: IC3.16 250.82,60.33 227.97,60.33 227.33,59.69 v223.52,59.69
N$6
  Route2 0.305: IC4.18 34.29,66.04 55.88,66.04 56.52,65.41 56.52,56.52 55.24,55.24 55.24,37.47 57.15,35.56 59.69,35.56 JP3.1
  Bottom 0.305: JP4.1 JP3.1
N$7  (via drill 0.6)
  Top 0.305: v215.9,40.64 v215.9,44.45
  Bottom 0.305: IC35.17 174.62,45.72 175.9,44.45 180.34,44.45 181.61,43.18 193.04,43.18 194.31,44.45 214.63,44.45 v215.9,44.45 | IC22.19 245.11,40.01 244.47,40.64 v215.9,40.64
N$8
  Top 0.305: LED1.K 158.75,12.06 161.29,9.53 R2.1
N$9
  Top 0.305: LED2.K 128.27,12.06 130.81,9.53 R3.1
N$10
  Top 0.305: LED3.K 100.33,10.16 R5.1
N$11
  Bottom 0.305: LED4.K R6.1
N$12
  Bottom 0.305: LED5.K R7.1
N$13
  Bottom 0.305: LED6.K R9.1
N$14
  Bottom 0.305: LED7.K R10.1
N$15
  Top 0.305: R11.1 LED8.K
N$16  (via drill 0.6)
  Route2 0.305: LED6.A 161.93,100.97 202.56,100.97 205.1,98.42 212.09,98.42 215.26,95.25 234.95,95.25 v235.59,95.89
  Route3 0.305: v235.59,95.89 v235.59,59.05
  Bottom 0.305: IC3.15 252.73,59.69 236.22,59.69 v235.59,59.05
N$17  (via drill 0.6)
  Route2 0.305: LED5.A 163.83,109.22 165.74,111.12 209.55,111.12 211.46,109.22 v222.25,109.22
  Route3 0.305: v222.25,109.22 222.25,107.95 220.98,106.68 v220.98,64.77
  Bottom 0.305: IC3.12 262.89,62.87 262.25,63.5 222.25,63.5 v220.98,64.77
N$18
  Top 0.305: IC35.3 179.71,48.26 180.97,49.53 180.97,51.44 181.61,52.07 SV1.8
  Bottom 0.305: SV1.8 RN9.2 | IC35.3 177.16,48.26 175.9,46.99 165.1,46.99 163.83,45.72 IC20.17
N$19  (via drill 0.6)
  Route2 0.305: LED4.A 160.02,100.33 201.93,100.33 204.47,97.79 211.46,97.79 216.53,92.71 222.88,92.71 v225.43,90.17
  Route3 0.305: v225.43,90.17 v225.43,66.04
  Bottom 0.305: IC3.9 262.89,67.94 261.62,66.67 226.06,66.67 v225.43,66.04
N$20  (via drill 0.6)
  Top 0.305: v212.72,66.04 212.09,65.41 212.09,13.34 v211.46,12.7
  Route2 0.305: LED3.A 102.23,14.61 169.23,14.61 169.86,13.97 203.84,13.97 205.1,12.7 v211.46,12.7
  Bottom 0.305: IC3.6 255.27,67.94 254.63,67.31 215.26,67.31 214,66.04 v212.72,66.04
N$21  (via drill 0.6)
  Top 0.305: v213.36,67.31 214,66.67 214,65.41 212.72,64.14 212.72,12.06 211.46,10.79 v211.46,8.89
  Route2 0.305: LED2.A 138.43,12.7 140.97,10.16 151.76,10.16 153.03,11.43 156.84,11.43 157.48,10.79 166.69,10.79 167.32,11.43 202.25,11.43 204.79,8.89 v211.46,8.89
  Bottom 0.305: IC3.5 252.73,68.58 252.09,67.94 214,67.94 v213.36,67.31
N$22  (via drill 0.6)
  Top 0.305: v211.46,69.22 211.46,14.29 210.19,13.02 v210.19,10.79
  Route2 0.305: LED1.A 202.88,12.7 205.42,10.16 206.69,10.16 207.33,10.79 v210.19,10.79
  Bottom 0.305: IC3.2 245.11,69.22 244.47,68.58 212.09,68.58 v211.46,69.22
N$23
  Bottom 0.305: R12.1 LED9.K
N$24
  Top 0.305: R13.1 69.85,8.26 67.31,10.79 LED10.K
N$25  (via drill 0.6)
  Top 0.305: JP8.1 96.52,34.29 92.71,38.1 92.71,67.94 90.81,69.85 v90.81,70.48
  Route2 0.305: IC7.18 105.41,69.22 104.78,69.85 91.44,69.85 v90.81,70.48
  Bottom 0.305: JP7.1 JP8.1
N$26
  Route2 0.305: IC4.16 36.83,67.94 38.1,66.67 56.52,66.67 57.15,66.04 57.15,55.88 55.88,54.61 55.88,39.37 57.15,38.1 59.69,38.1 JP3.2
  Bottom 0.305: JP4.2 JP3.2
N$27
  Route2 0.305: IC4.14 43.18,67.31 57.15,67.31 57.78,66.67 57.78,55.56 56.52,54.29 56.52,41.27 57.15,40.64 59.69,40.64 JP3.3
  Bottom 0.305: JP4.3 JP3.3
N$28
  Route2 0.305: IC4.12 48.26,69.85 57.78,69.85 58.42,69.22 58.42,55.24 57.15,53.98 57.15,43.81 57.78,43.18 60.33,43.18 60.96,42.55 JP3.4
  Bottom 0.305: JP4.4 JP3.4
N$29  (via drill 0.6)
  Top 0.305: v36.2,134.62 37.47,133.35 37.47,125.73 31.75,120.02 31.75,113.35 30.48,112.08 30.48,105.41 P8.8
  Bottom 0.305: IC1.21 66.67,133.35 65.41,132.08 61.59,132.08 61.28,132.4 51.75,132.4 49.53,134.62 v36.2,134.62
N$30
  Route2 0.305: IC4.9 48.26,74.93 58.42,74.93 59.05,74.3 59.05,55.88 64.77,50.16 64.77,45.72 66.04,44.45 JP4.5
  Bottom 0.305: JP4.5 JP3.5
N$31  (via drill 0.6)
  Top 0.305: v36.83,137.16 35.56,137.16 34.92,136.53 34.92,133.35 36.2,132.08 36.2,125.73 31.11,120.65 31.11,114.3 27.94,111.12 27.94,105.41 P8.7
  Bottom 0.305: IC1.22 61.28,135.89 60.33,134.94 52.39,134.94 50.16,137.16 v36.83,137.16
N$32
  Route2 0.305: IC4.7 43.18,77.47 58.42,77.47 59.69,76.2 59.69,56.2 65.41,50.48 65.41,47.62 66.04,46.99 JP4.6
  Bottom 0.305: JP4.6 JP3.6
N$33  (via drill 0.6)
  Top 0.305: v37.47,139.7 38.1,139.06 38.1,125.09 32.38,119.38 32.38,113.67 33.02,113.03 33.02,102.87 31.75,101.6 P8.6
  Bottom 0.305: IC1.23 64.14,138.43 62.23,140.34 50.16,140.34 49.53,139.7 v37.47,139.7
N$34
  Route2 0.305: IC4.5 36.83,76.83 38.1,78.11 58.74,78.11 60.33,76.52 60.33,56.52 66.04,50.8 66.04,50.16 66.67,49.53 JP4.7
  Bottom 0.305: JP4.7 JP3.7
N$35  (via drill 0.6)
  Top 0.305: v28.57,119.38 28.57,118.43 24.77,114.62 24.77,95.89 25.4,95.25 27.94,95.25 P8.2
  Bottom 0.305: IC2.23 v28.57,119.38
N$36
  Route2 0.305: IC4.3 31.75,77.47 33.02,78.74 59.05,78.74 60.96,76.83 60.96,56.83 63.18,54.61 64.96,52.9 65.79,52.07 JP4.8
  Bottom 0.305: JP4.8 JP3.8
N$37  (via drill 0.6)
  Top 0.305: v33.34,118.11 33.66,117.79 33.66,99.06 32.38,97.79 27.94,97.79 P8.3
  Bottom 0.305: IC2.22 34.61,116.84 v33.34,118.11
N$38  (via drill 0.6)
  Top 0.305: U5.A0 68.58,22.23 67.31,23.5 67.31,27.3 64.77,29.84 64.77,53.02 60.96,56.83 60.96,81.6 61.59,82.23 61.59,84.77 v61.28,85.09
  Bottom 0.305: IC5.18 31.75,81.28 34.29,83.82 56.52,83.82 57.78,85.09 v61.28,85.09
N$39
  Top 0.305: IC35.5 180.34,44.45 180.34,46.99 SV1.7
  Bottom 0.305: SV1.7 RN9.3 | IC35.5 177.16,43.18 175.9,41.91 166.37,41.91 165.1,40.64 IC20.15
N$40  (via drill 0.6)
  Top 0.305: U5.A1 66.04,22.23 64.77,23.5 64.77,26.67 64.14,27.3 64.14,52.7 60.33,56.52 60.33,81.92 60.64,82.23 v60.64,83.82
  Bottom 0.305: IC5.16 36.83,81.92 38.1,83.19 57.78,83.19 58.42,83.82 v60.64,83.82
N$41  (via drill 0.6)
  Top 0.305: U5.A2 63.5,22.23 62.23,23.5 62.23,26.67 63.5,27.94 63.5,52.39 59.69,56.2 59.69,80.01 59.37,80.33 v59.37,82.55
  Bottom 0.305: IC5.14 41.91,81.28 43.18,82.55 v59.37,82.55
N$42  (via drill 0.6)
  Top 0.305: U5.A3 60.96,22.23 59.69,23.5 59.69,27.3 62.87,30.48 62.87,52.07 59.05,55.88 59.05,79.06 58.42,79.69 v58.42,81.28
  Bottom 0.305: IC5.12 46.99,81.28 47.62,81.92 57.78,81.92 v58.42,81.28
N$43  (via drill 0.6)
  Top 0.305: U5.A4 58.42,22.23 57.15,23.5 57.15,27.94 56.52,28.57 56.52,53.34 58.42,55.24 58.42,75.88 57.47,76.83 57.47,82.87 60.33,85.72 60.33,87.63 59.69,88.27 v56.52,88.27
  Bottom 0.305: IC5.9 46.99,87 47.62,86.36 53.98,86.36 55.88,88.27 v56.52,88.27
N$44  (via drill 0.6)
  Top 0.305: U5.A5 55.88,22.23 54.61,23.5 54.61,27.3 55.88,28.57 55.88,53.66 57.78,55.56 57.78,75.56 56.83,76.52 56.83,83.19 59.05,85.41 v59.05,87
  Bottom 0.305: IC5.7 41.91,87 43.18,85.72 54.29,85.72 55.88,87.31 58.74,87.31 v59.05,87
N$45  (via drill 0.6)
  Top 0.305: U5.A6 53.34,22.23 52.07,23.5 52.07,26.04 55.24,29.21 55.24,53.98 57.15,55.88 57.15,74.93 56.2,75.88 56.2,83.5 57.15,84.45 v57.15,86.36
  Bottom 0.305: IC5.5 36.83,87 38.73,85.09 54.61,85.09 55.88,86.36 v57.15,86.36
N$46  (via drill 0.6)
  Top 0.305: v28.57,115.57 25.4,112.39 25.4,100.97 26.04,100.33 27.94,100.33 P8.4
  Bottom 0.305: IC2.21 38.1,114.3 36.83,115.57 v28.57,115.57
N$47  (via drill 0.6)
  Top 0.305: v31.75,111.76 31.75,104.14 30.48,102.87 27.94,102.87 P8.5
  Bottom 0.305: IC2.20 38.1,111.76 36.83,113.03 33.02,113.03 v31.75,111.76
N$48  (via drill 0.6)
  Top 0.635: P8.18 32.13,136.14 33.66,134.62 33.66,127 30.48,123.83 28.57,123.83 26.04,121.28 v26.04,118.11
  Bottom 0.635: v26.04,118.11 24.13,118.11 23.5,117.47 23.5,113.03 18.41,107.95 15.85,107.95 P2.1
N$49  (via drill 0.6)
  Top 0.635: P8.16 31.5,133.6 32.38,132.72 32.38,127.64 30.48,125.73 28.57,125.73 24.77,121.92 v24.77,116.2
  Bottom 0.635: P2.2 16.35,103.98 24.77,112.39 v24.77,116.2
N$50  (via drill 0.6)
  Top 0.305: U5.A7 50.8,20.95 49.53,22.23 49.53,25.4 54.61,30.48 54.61,54.29 56.52,56.2 56.52,74.3 55.56,75.25 55.56,84.45 v55.88,84.77
  Bottom 0.305: IC5.3 31.75,85.72 33.02,84.45 55.56,84.45 v55.88,84.77
N$51
  Top 0.305: RN14.2 69.85,22.86 69.85,19.05 U5.K0
N$52
  Top 1.422: D4.C 13.97,80.01 15.24,81.28 15.24,90.17 13.97,91.44 D3.A
  Bottom 1.422: P1.1 7.13,125.24
  Bottom 1.778: P1.2 10.34,128.24 P1.1 | 7.13,125.24 3.81,121.92 3.81,95.25 7.62,91.44 D3.A
N$53  (via drill 0.6)
  Top 0.305: JP8.2 96.52,36.83 93.34,40.01 93.34,69.85 v90.81,72.39
  Route2 0.305: IC7.16 110.49,69.22 109.22,70.48 92.71,70.48 v90.81,72.39
  Bottom 0.305: JP7.2 JP8.2
N$54
  Top 0.305: RN14.3 66.04,23.5 67.31,22.23 67.31,19.68 66.04,18.41 U5.K1
N$55  (via drill 0.6)
  Top 0.635: P8.14 30.23,131.06 31.11,130.18 31.11,128.27 29.84,127 27.94,127 v26.35,125.41
  Bottom 0.635: P2.3 12.38,103.19 13.34,102.23 20.32,102.23 23.5,105.41 23.5,107.31 27.3,111.12 27.3,124.46 v26.35,125.41
N$56
  Top 0.305: RN14.4 63.5,23.5 64.77,22.23 64.77,19.68 63.5,18.41 U5.K2
N$57
  Top 0.305: RN14.5 60.96,23.5 62.23,22.23 62.23,19.68 60.96,18.41 U5.K3
N$58
  Top 0.305: RN14.6 58.42,23.5 59.69,22.23 59.69,19.68 58.42,18.41 U5.K4
N$59
  Top 0.305: RN14.7 55.88,23.5 57.15,22.23 57.15,19.68 55.88,18.41 U5.K5
N$60
  Top 0.305: RN14.8 53.34,23.5 54.61,22.23 54.61,19.68 53.34,18.41 U5.K6
N$61
  Top 0.305: RN14.9 50.8,23.5 52.07,22.23 52.07,19.68 50.8,18.41 U5.K7
N$62  (via drill 0.6)
  Top 0.305: JP8.3 96.52,39.37 93.98,41.91 93.98,65.41 93.98,66.67 93.98,71.12 v92.71,72.39
  Route2 0.305: IC7.14 115.57,69.85 114.3,71.12 93.98,71.12 v92.71,72.39
  Bottom 0.305: JP7.3 JP8.3
N$63
  Top 0.305: IC5.17 34.29,78.74 33.02,77.47 33.02,73.66 34.29,72.39 IC4.17 35.56,67.31 35.56,54.61 34.29,53.34 34.29,50.8 IC33.19
N$64
  Top 0.305: IC5.15 39.37,78.74 38.1,77.47 38.1,73.66 39.37,72.39 IC4.15 39.37,67.31 38.1,66.04 38.1,55.24 37.47,54.61 37.47,42.55 36.83,41.91 IC33.16
N$65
